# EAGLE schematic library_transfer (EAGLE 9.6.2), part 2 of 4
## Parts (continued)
Unconnected: A1.1(AUD_ON) A1.3(AF_OUT) A1.5(PTT) A1.6(PD) A1.7(H/L) A1.8(VIN) A1.9(GND) A1.10(GND) A1.12(ANT) A1.16(RXD) A1.17(TXD) A1.18(MIC_IN) A2.P$1(GND1) A2.P$2(MISO) A2.P$3(MOSI) A2.P$4(SCK) A2.P$5(NSS) A2.P$6(RST) A2.P$7(DIO5) A2.P$8(GND2) A2.P$9(ANT) A2.P$10(GND3) A2.P$11(DIO3) A2.P$12(DIO4) A2.P$13(3.3V) A2.P$14(DIO0) A2.P$15(DIO1) A2.P$16(DIO2) A3.1(VIN+) A3.2(VIN-) A3.4(VOUT-) A3.6(VOUT+) A4.1(1-2) A4.2(1-2) A4.3(3-4) A4.4(3-4) A4.6 A4.7 A4.8 ANT1.P$1(GND) ANT1.P$2(ANT) ANT1.P$3(GND) ANT2.IN1 ANT3.IN1 ANT3.IN2 B1.1(P) B1.2(M) B1.3(N) B2.1(N) B2.2(M) B2.3(P) B3.+ B3.- B4.+1 B4.+2 B4.-1 B4.-2 B5.+1(+) B5.+2(+) B5.- B6.+ B6.- B7.N(-) B7.P(+) B8.+1(+) B8.+2(+) B8.-1(-) B8.-2(-) B11.+ B11.- B12.+ B12.- B13.N B13.P B14.+ B14.- B15.+ B15.- B16.1 B16.2 B17.+1(+) B17.+2(+) B17.-1(-) B17.-2(-) C1.P$1 C1.P$2 C2.+ C2.- C3.+ C3.- C4.P$1 C4.P$2 C5.+ C5.- C6.+ C6.- C7.P$1 C7.P$2 C8.P$1 C8.P$2 C9.1 C9.2 C10.P$1 C10.P$2 C11.COLD C11.HOT C12.COLD C12.HOT C13.+1 C13.+2 C13.-1 C13.-2 C14.N(-) C14.P(+) C15.+ C15.- C16.N(-) C16.P(+) C17.N(-) C17.P(+) C18.1A C18.1B C18.2A C18.2B C19.P$1 C19.P$2 C20.+ C20.- C21.+ C21.- C22.1 C22.2 C23.1 C23.2 C24.1 C24.2 C25.P$1 C25.P$2 C26.1 C26.2 C27.1 C27.2 C28.P$1 C28.P$2 C29.+ C29.- C30.+ C30.- C31.N(-) C31.P(+) C32.P$1 C32.P$2 CM1.1(GND) CM1.2(EMMC_DISABLE_N) CM1.3(GPIO-00) CM1.4(SDX_VDD) CM1.5(GPIO-01) CM1.6(SDX_VDD) CM1.7(GND) CM1.8(GND) CM1.9(GPIO-02) CM1.10(SDX_CLK) CM1.11(GPIO-03) CM1.12(SDX_CMD) CM1.13(GND) CM1.14(GND) CM1.15(GPIO-04) CM1.16(SDX_D0) CM1.17(GPIO-05) CM1.18(SDX_D1) CM1.19(GND) CM1.20(GND) CM1.21(GPIO-06) CM1.22(SDX_D2) CM1.23(GPIO-07) CM1.24(SDX_D3) CM1.25(GND) CM1.26(GND) CM1.27(GPIO-08) CM1.28(GPIO-28) CM1.29(GPIO-09) CM1.30(GPIO-29) CM1.31(GND) CM1.32(GND) CM1.33(GPIO-10) CM1.34(GPIO-30) CM1.35(GPIO-11) CM1.36(GPIO-31) CM1.37(GND) CM1.38(GND) CM1.39(GPIO0-27_VDD) CM1.40(GPIO0-27_VDD) CM1.41(GPIO28-45_VDD) CM1.42(GPIO28-45_VDD) CM1.43(GND) CM1.44(GND) CM1.45(GPIO-12) CM1.46(GPIO-32) CM1.47(GPIO-13) CM1.48(GPIO-33) CM1.49(GND) CM1.50(GND) CM1.51(GPIO-14) CM1.52(GPIO-34) CM1.53(GPIO-15) CM1.54(GPIO-35) CM1.55(GND) CM1.56(GND) CM1.57(GPIO-16) CM1.58(GPIO-36) CM1.59(GPIO-17) CM1.60(GPIO-37) CM1.61(GND) CM1.62(GND) CM1.63(GPIO-18) CM1.64(GPIO-38) CM1.65(GPIO-19) CM1.66(GPIO-39) CM1.67(GND) CM1.68(GND) CM1.69(GPIO-20) CM1.70(GPIO-40) CM1.71(GPIO-21) CM1.72(GPIO-41) CM1.73(GND) CM1.74(GND) CM1.75(GPIO-22) CM1.76(GPIO-42) CM1.77(GPIO-23) CM1.78(GPIO-43) CM1.79(GND) CM1.80(GND) CM1.81(GPIO-24) CM1.82(GPIO-44) CM1.83(GPIO-25) CM1.84(GPIO-45) CM1.85(GND) CM1.86(GND) CM1.87(GPIO-26) CM1.88(HDMI_HPD_N_1V8) CM1.89(GPIO-27) CM1.90(EMMC_EB_N_1V8) CM1.91(GND) CM1.92(GND) CM1.93(DSI0_DN1) CM1.94(DSI1_DP0) CM1.95(DSI0_DP1) CM1.96(DSI1_DN0) CM1.97(GND) CM1.98(GND) CM1.99(DSI0_DN0) CM1.100(DSI1_CP) CM1.101(DSI0_DP0) CM1.102(DSI1_CN) CM1.103(GND) CM1.104(GND) CM1.105(DSI0_CN) CM1.106(DSI1_DP3) CM1.107(DSI0_CP) CM1.108(DSI1_DN3) CM1.109(GND) CM1.110(GND) CM1.111(HDMI_CLK_N) CM1.112(DSI1_DP2) CM1.113(HDMI_CLK_P) CM1.114(DSI1_DN2) CM1.115(GND) CM1.116(GND) CM1.117(HDMI_D0_N) CM1.118(DSI1_DP1) CM1.119(HDMI_D0_P) CM1.120(DSI1_DN1) CM1.121(GND) CM1.122(GND) CM1.123(HDMI_D1_N) CM1.124(NC) CM1.125(HDMI_D1_P) CM1.126(NC) CM1.127(GND) CM1.128(NC) CM1.129(HDMI_D2_N) CM1.130(NC) CM1.131(HDMI_D2_P) CM1.132(NC) CM1.133(GND) CM1.134(GND) CM1.135(CAM1_DP3) CM1.136(CAM0_DP0) CM1.137(CAM1_DN3) CM1.138(CAM0_DN0) CM1.139(GND) CM1.140(GND) CM1.141(CAM1_DP2) CM1.142(CAM0_CP) CM1.143(CAM1_DN2) CM1.144(CAM0_CN) CM1.145(GND) CM1.146(GND) CM1.147(CAM1_CP) CM1.148(CAM0_DP1) CM1.149(CAM1_CM) CM1.150(CAM0_DN1) CM1.151(GND) CM1.152(GND) CM1.153(CAM1_DP1) CM1.154(NC) CM1.155(CAM1_DN1) CM1.156(NC) CM1.157(GND) CM1.158(NC) CM1.159(CAM1_DP0) CM1.160(NC) CM1.161(CAM1_DN0) CM1.162(NC) CM1.163(GND) CM1.164(GND) CM1.165(USB_DP) CM1.166(TVDAC) CM1.167(USB_DN) CM1.168(USB_OTGID) CM1.169(GND) CM1.170(GND) CM1.171(HDMI_CEC) CM1.172(VC_TRST_N) CM1.173(HDMI_SDA) CM1.174(VC_TDI) CM1.175(HDMI_SCL) CM1.176(VC_TMS) CM1.177(RUN) CM1.178(VC_TDO) CM1.179(VDD_CORE_(DNC)) CM1.180(VC_TCK) CM1.181(GND) CM1.182(GND) CM1.183(1.8V) CM1.184(1.8V) CM1.185(1.8V) CM1.186(1.8V) CM1.187(GND) CM1.188(GND) CM1.189(VDAC) CM1.190(VDAC) CM1.191(3.3V) CM1.192(3.3V) CM1.193(3.3V) CM1.194(3.3V) CM1.195(GND) CM1.196(GND) CM1.197(VBATT) CM1.198(VBATT) CM1.199(VBATT) CM1.200(VBATT) CR1.A CR1.C(K) CR2.1(K) CR2.2(A) CR3.A CR3.C(K) CR4.1(A) CR4.2(A) CR4.3(K) CR5.1(A1) CR5.2(K) CR5.3(A2) CR6.1 CR6.3 CR6.TAB CR7.A CR7.K CR8.A CR8.K CR9.A CR9.C(K) CR10.A CR10.C(K) CR11.1(A1) CR11.3(A2) CR11.T(K) CR12.A CR12.K CR13.P$1 CR13.P$2 CR13.P$3 CR14.1 CR14.3 CR14.TAB CR15.1 CR15.2 CR15.3 CR16.A CR16.K CR17.A CR17.K CR18.1(K) CR18.2(A) CR19.1(K) CR19.2(A) CR20.A CR20.C(K) CR21.A CR21.C(K) CR22.A CR22.K D1.A1 D1.A2 D1.K1 D1.K2 D2.A D2.K D3.A D3.K1(K) D3.K2(K) D4.1(K) D4.3(A) D5.A D5.K D6.1(A) D6.2(K) D7.2(GND) D7.3(VCC) D7.4(IO2) D7.5(IO1) D8.1(A) D8.2(K) D8.3(COM) D9.A D9.C(K) D10.A D10.K D11.A D11.K D12.1(CC1) D12.2(E) D12.3(D) D12.4(C) D12.5(CC2) D12.6(B) D12.7(A) D12.8(DP) D12.9(F) D12.10(G) D13.A D13.K D14.1(K) D14.3(A) D15.1(A) D15.3(A) D15.T(K) D16.A D16.K D17.A D17.K D18.1(K) D18.2(A) D19.1(K) D19.2(A) D20.1(K) D20.2(A) D21.A D21.K1(K) D21.K2(K) D22.1(A) D22.2(A) D22.3(K) D23.A D23.K D24.A D24.K D25.1(REF) D25.2(K) D25.3(A) D26.1(A) D26.3(K) D27.A D27.K(C) D28.A D28.K D29.A D29.K(C) D30.A D30.K D31.A D31.K(C) D32.A D32.K D33.A D33.K D34.A D34.C(K) D35.A D35.K D36.1(K) D36.2(A) F1.P$1 F1.P$2 F2.P$1 F2.P$2 F3.P$1 F3.P$2 F4.P$1 F4.P$2 F5.P$1 F5.P$2 F6.P$1 F6.P$2 F7.P$1 F7.P$2 F8.1 F8.2(GND) F8.3(GND) F8.4 F8.5(GND) F9.P$1 F9.P$2 F10.1A F10.2A F10.3B F10.4B F13.P$1 F13.P$2 F14.P$1 F14.P$2 F15.P$1 F15.P$2 F16.P$1 F16.P$2 FB1.P$1 FB1.P$2 GDT1.P$1 GDT1.P$2 GDT2.P$1 GDT2.P$2 GDT3.C GDT3.L1 GDT3.L2 HS1.P$1 HS1.P$2 HS1.P$3 HS1.P$4 HS2.P$1 HS2.P$2 HS3.P$1 HS3.P$2 HS4.P$1 HS4.P$2 HS4.P$3 HS4.P$4 HS5.P$1 HS5.P$2 J1.1 J1.2 J1.3 J1.4 J2.N J2.P J3.+(P) J3.-(N) J4.+(P) J4.-(N) J5.N J5.P J6.+(P) J6.-(N) J7.A1(GND) J7.A4(VCC) J7.A5(CC1) J7.A6(D+) J7.A7(D-) J7.A8(SBV1) J7.A9(VCC) J7.A12(GND) J7.B1(GND) J7.B4(VCC) J7.B5(CC2) J7.B6(D+) J7.B7(D-) J7.B8(SBV2) J7.B9(VCC) J7.B12(GND) J8.A1(GND) J8.A4(VCC) J8.A5(CC1) J8.A6(D+) J8.A7(D-) J8.A8(SBV1) J8.A9(VCC) J8.A12(GND) J8.B1(GND) J8.B4(VCC) J8.B5(CC2) J8.B6(D+) J8.B7(D-) J8.B8(SBV2) J8.B9(VCC) J8.B12(GND) J9.A1(GND) J9.A4(VCC) J9.A5(CC1) J9.A6(D+) J9.A7(D-) J9.A8(SBV1) J9.A9(VCC) J9.A12(GND) J9.B1(GND) J9.B4(VCC) J9.B5(CC2) J9.B6(D+) J9.B7(D-) J9.B8(SBV2) J9.B9(VCC) J9.B12(GND) J10.1(VCC1) J10.2(D-1) J10.3(D+1) J10.4(GND1) J10.5(VCC2) J10.6(D-2) J10.7(D+2) J10.8(GND2) J10.G1(CASE1) J10.G2(CASE1) J10.G3(CASE2) J10.G4(CASE2) J11.1(VCC) J11.2(D-) J11.3(D+) J11.4(GND) J11.S1(CASE) J11.S2(CASE) J12.1(VCC) J12.2(D-) J12.3(D+) J12.4(GND) J12.MH1(CASE) J12.MH2(CASE) J13.1(NC1) J13.2(NC2) J13.3(IN) J13.4(NC4) J13.5(NC5) J13.6(CAP) J13.7(NC7) J13.8(NC8) J13.9(NC9) J13.10(OUT10) J13.11(OUT11) J13.12(NC12) J13.13(NC13) J13.14(NC14) J13.15(NC15) J13.16(NC16) J13.EP J14.1A J14.1B J14.2A J14.2B J14.3A J14.3B J15.1A J15.1B J15.2A J15.2B J16.G1(GND) J16.G2(GND) J16.G3(GND) J16.G4(GND) J16.S(RF) J17.G1(GND) J17.G2(GND) J17.G3(GND) J17.G4(GND) J17.RF J18.1(S) J18.2(T) J18.3(R) J19.R J19.S J19.T J20.1(S) J20.2(T) J20.3(R) J21.R J21.S J21.T J22.1(S) J22.2(T) J22.3(R1) J22.4(R2) J23.P$1 J23.P$2 J24.1 J24.2 J24.3 J24.4 J24.5 J24.6 J24.7 J24.8 J24.9 J24.10 J25.DND4(GND) J25.GND1(GND) J25.GND2(GND) J25.GND3(GND) J25.SIG(RF) J26.C1(VSS) J26.C2(VSS) J26.C3(VSS) J26.C4(VSS) J26.DSW1(SW1) J26.DSW2(SW2) J26.P1(DAT2) J26.P2(DAT3/CS) J26.P3(CMD/MOSI) J26.P4(VDD) J26.P5(CLK) J26.P6(VSS) J26.P7(DAT0/MISO) J26.P8(DAT1) J27.1(D2) J27.2(D3) J27.3(CMD) J27.4(VDD) J27.5(CLK) J27.6(VSS) J27.7(D0) J27.8(D1) J27.P$1(CASE) J27.P$2(CASE) J27.P$3(CASE) J27.P$4(CASE) J28.1 J28.2 J28.3 J28.4 J28.5 J28.6 J28.7 J28.8 J28.9 J28.10 J28.11 J28.12 J28.13 J28.14 J28.15 J29.1 J29.2 J29.3 J29.4 J29.5 J29.6 J29.7 J29.8 J29.9 J30.1A J30.1B J30.2A J30.2B J30.3A J30.3B J31.1A J31.1B J31.2A J31.2B J32.1(V+) J32.2(GND) J32.3(NO) J33.G1(GND) J33.G2(GND) J33.SIG(RF) J34.GND1(GND) J34.GND2(GND) J34.GND3(GND) J34.GND4(GND) J34.RF J35.1 J35.2 J35.3 J35.4 J35.5 J35.6 J35.7 J35.8 J35.9 J35.10 J35.11 J35.12 J35.13 J35.14 J35.15 J35.16 J36.1 J36.2 J36.3 J36.4 J36.MECH1(MT1) J36.MECH2(MT2) J37.P$1 J38.1 J38.2 J38.3 J38.4 J38.5 J39.1 J39.2 J39.3 J39.4 J39.5 J39.6 J39.7 J39.8 J39.9 J39.10 J39.11 J39.12 J39.13 J39.14 J39.15 J39.16 J39.17 J39.18 J39.19 J39.20 J39.21 J39.22 J39.23 J39.24 J39.25 J39.26 J39.27 J39.28 J39.29 J39.30 J39.31 J39.32 J39.33 J39.34 J39.35 J39.36 J39.37 J39.38 J39.39 J39.40 J40.1(VCC1) J40.2(D-1) J40.3(D+1) J40.4(GND1) J40.5(VCC2) J40.6(D-2) J40.7(D+2) J40.8(GND2) J40.P$9(CASE1) J40.P$10(CASE2) J40.P$11(CASE2) J40.P$12(CASE1) J41.1(VCC) J41.2(D-) J41.3(D+) J41.4(GND) J41.P$5(CASE) J41.P$6(CASE) J42.1(RTH_TCT) J42.2(ETH_TDP) J42.3(ETH_TDN) J42.4(ETH_RDP) J42.5(USB_RDN) J42.6(ETH_RCT) J42.13(RIGHT_LED_C) J42.14(RIGHT_LED_A) J42.15(LEFT_LED_C) J42.16(LEFT_LED_A) J42.P$5(SHIELD) J42.P$6(SHIELD) J42.P$7(SHIELD) J42.P$8(SHIELD) J42.P$9(SHIELD) J42.P$10(SHIELD) J42.U1(USB_VCC) J42.U2(USB_DM) J42.U3(USB_DP) J42.U4(USB_GND) J43.1(NC) J43.2(AGND) J43.3(SDA) J43.4(AVDD) J43.5(SCL) J43.6(RESET) J43.7(VS) J43.8(PWDN) J43.9(HS) J43.10(DVDD) J43.11(DOVDD) J43.12(D9) J43.13(MCLK) J43.14(D8) J43.15(DGND) J43.16(D7) J43.17(PCLK) J43.18(D6) J43.19(D2) J43.20(D5) J43.21(D3) J43.22(D4) J43.23(D1) J43.24(D0) J43.P$1(DGND) J43.P$2(DGND) J44.P$1 J45.1 J45.2 J45.3 J45.4 J45.5 J45.6 J45.7 J45.8 J45.9 J46.1 J46.2 J46.3 J46.4 J46.5 J46.6 J46.7 J46.8 J46.9 J47.1 J47.2 J47.3 J47.4 J47.5 J47.6 J47.7 J47.8 J47.S1 J47.S2 J49.1A J49.1B J49.2A J49.2B J50.1 J50.2 J51.1 J51.2 J51.3 J51.4 J51.5 J52.G1(GND) J52.G2(GND) J52.G3(GND) J52.G4(GND) J52.S(RF) J53.P$1(RF) J53.P$2(GND) J53.P$3(GND) J53.P$4(GND) J53.P$5(GND) J54.N(GND) J54.P(RF) J54.S1(GND) J54.S2(GND) J55.1 J55.2 J56.1 J56.2 J56.3 J56.4 J56.5 J56.6 J56.7 J56.8 J56.9 J56.10 J56.11 J56.12 J56.13 J56.14 J56.15 J56.16 J56.17 J56.18 J56.19 J56.20 J56.21 J56.22 J56.23 J56.24 J56.25 J56.26 J56.27 J56.28 J56.29 J56.30 J56.31 J56.32 J56.33 J56.34 J56.35 J56.36 J56.37 J56.38 J56.39 J56.40 J56.FN1(FN) J56.FN2(FN) J56.FN3(FN) J56.FN4(FN) J57.1 J57.2 J58.1A J58.1B J58.2A J58.2B J58.3A J58.3B J58.4A J58.4B J58.5A J58.5B J58.6A J58.6B J58.7A J58.7B J58.8A J58.8B J59.L J59.R J60.1 J60.2 J60.3 J61.1 J61.2 J61.3 J62.1(1VCC) J62.2(2DM) J62.3(3DP) J62.4(4ID) J62.5(5GND) J62.GND(CASE) J63.1 J63.2 J63.3 J63.4 J63.5 J63.6 J63.7 J63.8 J63.9 J63.10 J63.11 J63.12 J63.13 J63.14 J63.15 J63.16 J63.17 J63.18 J63.19 J63.20 J63.21 J63.22 J63.23 J63.24 J63.25 J63.26 J63.27 J63.28 J63.29 J63.30 J63.31 J63.32 J63.33 J63.34 J63.35 J63.36 J63.37 J63.38 J63.39 J63.40 J63.41 J63.42 J63.43 J63.44 J63.45 J63.46 J63.47 J63.48 J63.49 J63.50 J63.51 J63.52 J63.53 J63.54 J63.55 J63.56 J63.57 J63.58 J63.59 J63.60 J63.61 J63.62 J63.63 J63.64 J64.1 J64.2 J64.3 J64.4 J64.5 J64.M1(C) J64.M2(C) J64.M3(C) J64.M4(C) J65.1 J65.2 J65.3 J65.4 J65.5 J65.6 J65.7 J65.8 J65.S1 J65.S2 J66.G1(GND) J66.G2(GND) J66.G3(GND) J66.G4(GND) J66.RF J67.1 J67.2 J68.1 J68.2 J68.P1 J68.P2 J69.P$1 J70.RING J70.TIP J71.1 J71.2 J71.3 J71.4 J71.5 J71.6 J72.P$1 J72.P$2 J72.P$3 J72.P$4 J72.P$5 J72.P$6 J72.P$7 J72.P$8 J73.P$1 J73.P$2 J73.P$3 J73.P$4 J73.P$5 J73.P$6 J74.P$1 J74.P$2 J74.P$3 J74.P$4 J75.P$1 J75.P$2 J76.P$1 J77.P$1 J78.P$1 J78.P$2 J78.P$3 J78.P$4 J79.P$1 J79.P$2 J79.P$3 J79.P$4 J80.GND J80.L J80.N J81.1 J81.2 J81.3 J81.4 J81.5 J81.6 J81.7 J81.8 J81.9 J81.10 J81.11 J81.12 J81.13 J81.14 J82.1(SHIELD_2) J82.2(DATA_2_P) J82.3(DATA_2_N) J82.4(SHIELD_1) J82.5(DATA_1_P) J82.6(DATA_1_N) J82.7(SHIELD_0) J82.8(DATA_0_P) J82.9(DATA_0_N) J82.10(SHIELD_CLK) J82.11(CLK_P) J82.12(CLK_N) J82.13(GND) J82.14(CEC) J82.15(SCL) J82.16(SDA) J82.17(UTILITY) J82.18(+5V) J82.19(HPD) J82.P$1(GND) J82.P$2(GND) J82.P$3(GND) J82.P$4(GND) J83.1(BTM) J83.2(BTM) J83.3(TOP) J84.1 J84.2 J85.1 J85.2 J85.3 J85.4 J85.5 J85.6 J85.7 J85.8 J85.9 J85.10 J85.11 J85.12 J85.13 J85.14 J85.15 J85.16 J85.17 J85.18 J85.19 J85.20 J86.P$1 J86.P$2 J87.1 J87.2 J87.3 J87.4 J87.5 J87.6 J87.7 J87.8 J87.9 J87.10 J88.1 J88.2 J88.3 J88.4 J88.5 J88.6 J88.7 J88.8 J88.9 J88.10 L1.P$1 L1.P$2 L2.P$1 L2.P$2 L3.P$1 L3.P$2 L4.P$1 L4.P$2 L5.P$1 L5.P$2 L6.P$1 L6.P$2 L7.P$1 L7.P$2 L8.P$1 L8.P$2 L9.P$1 L9.P$2 L10.P$1 L10.P$2 L11.P$1 L11.P$2 L12.P$1 L12.P$2 L13.P$1 L13.P$2 L14.P$1 L14.P$2 L15.P$1 L15.P$2 L16.P$1 L16.P$2 L17.IN1(1IN) L17.IN2(2IN) L17.OUT1(1OUT) L17.OUT2(2OUT) L18.P$1 L18.P$2 L19.1 L19.2 L20.1 L20.2 L21.A1(1IN) L21.A2(1OUT) L21.B1(2IN) L21.B2(2OUT) L22.1 L22.2 L23.P$1 L23.P$2 L24.1(P+) L24.3(P-) L24.4(S+) L24.5(SCT) L24.6(S-) L25.P$1 L25.P$2 L26.P$1 L26.P$2 L27.P$1 L27.P$2 L28.P$1 L28.P$2 L29.P$1 L29.P$2 L30.P$1 L30.P$2 L31.P$1 L31.P$2 L32.P$1 L32.P$2 L33.P$1 L33.P$2 L34.P$1 L34.P$2 L35.P$1 L35.P$2 L36.P$1 L36.P$2 L37.P$1 L37.P$2 L38.P$1 L38.P$2 L39.P$1 L39.P$2 L40.P$1 L40.P$2 L41.IN1(1IN) L41.IN2(2IN) L41.OUT1(1OUT) L41.OUT2(2OUT) L42.1 L42.2 L43.1(1IN) L43.2(2IN) L43.3(1OUT) L43.4(2OUT) L44.P$1 L44.P$2 L45.P$1 L45.P$2 L46.1(1IN) L46.2(2IN) L46.3(2OUT) L46.4(1OUT) L47.P$1 L47.P$2 L48.1 L48.2 L49.1(1IN) L49.2(1OUT) L49.3(2OUT) L49.4(2IN) L50.1(1IN) L50.2(1OUT) L50.3(2OUT) L50.4(2IN) L51.P$1 L51.P$2 L52.P$1 L52.P$2 L53.P$1 L53.P$2 L54.P$1 L54.P$2 L55.P$1 L55.P$2 L56.P$1 L56.P$2 L57.P$1 L57.P$2 L58.1 L58.2 L59.1 L59.2 L60.P$1 L60.P$2 L61.P$1 L61.P$2 L62.1 L62.2 LS1.P$1 LS1.P$2 MOV1.P$1 MOV1.P$2 Q1.1(B) Q1.3(E) Q1.T(C) Q2.1(G) Q2.2(S) Q2.3(D) Q3.1(G) Q3.2(D) Q3.3(S) Q4.1(S) Q4.2(S) Q4.3(S) Q4.4(G) Q4.5(D) Q4.6(D) Q4.7(D) Q4.8(D) Q5.1(G) Q5.2(D) Q5.3(S) Q5.T(D) Q6.1(S) Q6.2(S) Q6.3(S) Q6.4(G) Q6.15(D) Q7.1_S(S) Q7.2_S(S) Q7.3_S(S) Q7.4_G(G) Q7.5_D(D) Q7.6_D(D) Q7.7_D(D) Q7.8_D(D) Q7.D Q8.1(S) Q8.2(S) Q8.3(S) Q8.4(G) Q8.15(D) Q10.1(G) Q10.3(S) Q10.TAB(D) Q11.D Q11.G Q11.S Q12.1(B) Q12.2(E) Q12.3(C) Q13.1(B) Q13.2(E) Q13.3(C) Q14.1(G) Q14.3(S) Q14.TAB(D) Q15.1(B) Q15.2(E) Q15.3(C) Q16.1(B) Q16.2(E) Q16.3(C) Q17.1(B) Q17.2(E) Q17.3(C) Q18.1(G) Q18.3(S) Q18.T(D) Q19.1(G) Q19.3(S) Q19.T(D) Q20.1(G) Q20.2(D) Q20.3(S) Q21.1(G) Q21.2(D) Q21.3(S) Q22.1(G) Q22.3(S) Q22.TAB(D) Q23.1(G) Q23.2(D) Q23.3(S) Q24.1(G) Q24.3(S) Q24.T(D) Q25.D Q25.G Q25.S Q26.1(S) Q26.2(S) Q26.3(S) Q26.4(G) Q26.5(D) Q26.6(D) Q26.7(D) Q26.8(D) Q26.P$1(D) Q27.1(S) Q27.2(S) Q27.3(S) Q27.4(G) Q27.5(D) Q27.6(D) Q27.7(D) Q27.8(D) Q27.8_P(D) Q28.1(S) Q28.2(G) Q28.3(D) Q28.4(S) Q28.5(G) Q28.6(D) Q29.1(G) Q29.2(D) Q29.3(S) Q29.4(S) Q29.5(D) Q29.6(D) Q29.7(S) Q29.8(S) Q29.9(D) Q29.10(D) Q29.11(S) Q29.12(S) Q29.13(D) Q29.14(D) Q29.15(S) Q29.16(S) Q29.17(D) Q29.18(D) Q29.19(S) Q29.20(S) Q29.21(D) Q29.22(D) Q29.23(S) Q29.24(S) Q29.25(D) Q29.26(D) Q29.27(S) Q29.28(S) Q29.29(D) Q29.30(D) Q30.1(G) Q30.2(S) Q30.3(D) Q31.D Q31.G Q31.S Q32.1(VIN) Q32.3(TG) Q32.4(TGR) Q32.5(BG) Q32.6(SW) Q32.7(SW) Q32.8(SW) Q32.TP(PGND) Q33.1(S) Q33.2(S) Q33.3(S) Q33.4(G) Q33.5(D) Q33.6(D) Q33.7(D) Q33.8(D) Q33.TP(D) Q34.1(D) Q34.2(D) Q34.3(G) Q34.4(S) Q34.5(D) Q34.6(D) Q34.7(S) Q34.8(D) Q35.1(G) Q35.2(D) Q35.3(S) Q35.T(D) Q36.D1(D) Q36.D2(D) Q36.D3(D) Q36.G Q36.S Q37.1(G) Q37.2(S) Q37.3(D) Q38.1(D) Q38.2(G) Q38.3(S) Q38.4(G) Q38.5(D) Q38.6(S) Q39.1(S) Q39.2(S) Q39.3(S) Q39.4(G) Q39.5(D) Q39.6(D) Q39.7(D) Q39.8(D) Q40.1(G) Q40.2(S) Q40.3(D) Q41.1(G) Q41.2(D) Q41.G(S) Q42.D Q42.G Q42.P$2(S) Q42.P$3(S) Q42.S Q43.D Q43.G Q43.S R1.1 R1.2 R2.1 R2.2(ADJ) R2.3 R3.1 R3.2(ADJ) R3.3 R4.1 R4.2 R4.3 R5.1 R5.2 R5.3 R6.1 R6.2 R6.3 R7.1 R7.2 R7.3 R8.1 R8.2 R8.3 R9.1 R9.2 R9.3 R9.S1 R9.S2 R10.P$1 R10.P$2 R11.1 R11.2 R11.3 R12.1 R12.2 R13.1 R13.2 R14.1 R14.2 R15.1 R15.2 RT1.1 RT1.2 S2.1 S2.7 S2.8(NO) S2.9(GND) S2.10(GND) S2.11(COM) S2.12(GND) S2.13(GND) S2.14(NC) S3.P$1 S3.P$2 S3.P$3 S3.P$4 S3.P$5 S3.P$6 S3.P$7 S3.P$8 S3.P$9 S3.P$10 S3.P$11 S3.P$12 S3.P$13 S3.P$14 S3.P$15 S3.P$16 S3.P$17 S3.P$18 S3.P$19 S3.P$20 S3.P$21 S3.P$22 S3.P$23 S3.P$24 S3.P$25 S3.P$26 S3.P$27 S3.P$28 SH1.P$1 SH1.P$2 SH1.P$3 SH1.P$4 SH1.P$5 SH1.P$6 SH1.P$7 SH1.P$8 SH1.P$9 SH1.P$10 SH1.P$11 SH1.P$12 SW1.1 SW1.2 SW1.3 SW1.4 SW1.C SW2.1 SW2.2 SW2.A SW2.B SW2.C SW3.S1 SW3.S2 SW4.SW1 SW4.SW2 SW5.1 SW5.2 SW5.3 SW5.4 SW5.5 SW5.7 SW5.8 SW5.9 SW5.10 SW5.11 SW5.A SW5.B SW6.C(COM) SW6.L SW6.R SW7.1 SW7.2(COM) SW7.3 SW8.C(COM) SW8.L SW8.R SW9.1 SW9.2 SW9.C(COM) SW10.1 SW10.2 SW10.3 SW10.4 SW10.5 SW10.6 T1.P$1 T3.1(OUT+) T3.2(GND2) T3.3(OUT-) T3.4(IN) T3.5(GND1) T4.1(1P_PHY) T4.2(1C_PHY) T4.3(1N_PHY) T4.6(2P_PHY) T4.7(2C_PHY) T4.8(2N_PHY) T4.9(2N) T4.10(2C) T4.11(2P) T4.14(1N) T4.15(1C) T4.16(1P) T5.1 T5.2 T5.3 T5.4 T5.5 T5.6 T6.1IN T6.1OUT T6.2IN T6.2OUT T7.1B T7.1F T7.2B T7.2F T8.1 T8.2 T8.3 T8.4 T8.5 T8.6 T9.1 T9.2 T9.3 T9.4 T9.5 T9.6 TP1.P$1 TP2.P$1 TP3.P$1 TP4.P$1 U1.1(V+) U1.2(IN) U1.3(GND) U1.4(SINK) U1.5(IN) U1.6(SOURCE) U2.1(GND) U2.2(OUT) U2.3(IN) U3.1(GND) U3.2(OUT) U3.3(IN) U4.1(GND1) U4.2(VCC) U4.3(DIO13/DOUT) U4.4(DIN/DIO14) U4.5(DIO12) U4.6(!RESET) U4.7(DIO10/RSSI) U4.8(DIO11/PWM1) U4.9(RSVD1) U4.10(DIO8/!DTR) U4.11(GND2) U4.12(DIO19/!SPI_ATTN) U4.13(GND3) U4.14(DIO18/SPI_CLK) U4.15(DIO17/!SPI_SS) U4.16(DIO16/SPI_MOSI) U4.17(DIO15/SPI_MISO) U4.18(RSVD2) U4.19(RSVD3) U4.20(RSVD4) U4.21(RSVD5) U4.22(GND4) U4.23(RSVD6) U4.24(DIO4) U4.25(DIO7/!CTS) U4.26(DIO9/!SLEEP) U4.27(VREF) U4.28(DIO5/ASSOC) U4.29(DIO6/!RTS) U4.30(DIO3/AD3) U4.31(DIO2/AD2) U4.32(DIO1/AD1) U4.33(DIO0/AD0) U4.34(RSVD7) U4.35(GND5) U4.36(RF) U4.37(RSVD8) U4.38(GND_PAD) U5.1(RST) U5.2(MISO) U5.3(MOSI) U5.4(SCK) U5.5(NSS) U5.6(VCC) U5.7(GND1) U5.8(NC) U5.9(GND2) U5.10(DIO1) U5.11(BUSY) U5.12(GND3) U5.13(GND4) U5.14(ANT) U6.1(+VIN) U6.2(ON/OFF) U6.3(-VIN) U6.4(-VOUT) U6.5(-SENSE) U6.6(TRIM) U6.7(+SENSE) U6.8(+VOUT) U7.1(IO1) U7.2(GND) U7.3(I02) U7.4(IO3) U7.5(VBUS) U7.6(IO4) U8.1(IN1) U8.2(IN2) U8.3(IN3) U8.4(IN4) U8.5(IN5) U8.6(IN6) U8.7(IN7) U8.8(GND) U8.9(VCC) U8.10(OUT7) U8.11(OUT6) U8.12(OUT5) U8.13(OUT4) U8.14(OUT3) U8.15(OUT2) U8.16(OUT1) U9.1(VDD) U9.2(GND) U9.3(IN+) U9.4(IN-) U9.5(OUT) U10.1(VDD) U10.2(HB) U10.3(HO) U10.4(HS) U10.5(HI) U10.6(LI) U10.7(VSS) U10.8(LO) U10.TP(VSS) U11.1(VCC) U11.2(OUT) U11.3(GND) U11.4(NC) U12.1(VCC) U12.2(X+) U12.3(Y+) U12.4(X-) U12.5(Y-) U12.6(GND) U12.7(VBAT) U12.8(AUX) U12.9(VREF) U12.10(IOVDD) U12.11(!PENIRQ) U12.12(DOUT) U12.13(BUSY) U12.14(DIN) U12.15(!CS) U12.16(DCLK) U13.1(OUT) U13.2(IN-) U13.3(IN+) U13.4(-VS) U13.5(IN+) U13.6(IN-) U13.7(OUT) U13.8(+VS) U14.1(NO) U14.2(GND) U14.3(NC) U14.4(COM) U14.5(VCC) U14.6(IN) U15.1(NO) U15.2(GND) U15.3(NC) U15.4(COM) U15.5(VCC) U15.6(IN) U16.1(IN) U16.2(GND) U16.3(EN) U16.5(OUT) U17.1(VOUT) U17.2(L2) U17.3(PGND) U17.4(L1) U17.5(VIN) U17.6(EN) U17.7(PS/SYNC) U17.8(VINA) U17.9(GND) U17.10(FB) U17.PG1(PGND) U17.PG2(PGND) U17.PG3(PGND) U17.PG4(PGND) U17.PG(PGND) U18.1(SW) U18.2(SW) U18.3(SW) U18.4(PG) U18.5(FB) U18.6(AGND) U18.7(FSW) U18.8(DEF) U18.9(SS) U18.10(AVIN) U18.11(PVIN) U18.12(PVIN) U18.13(EN) U18.14(VOS) U18.15(PGND) U18.16(PGND) U18.EP(PGND) U19.1(VIN) U19.2(CTRL) U19.3(SW) U19.4(GND) U19.5(COMP) U19.6(FB) U20.1(FSW) U20.2(VCC) U20.3(FB) U20.4(COMP) U20.5(GND) U20.6(VOUT) U20.7(EN) U20.8(ILIM) U20.9(VIN) U20.10(BOOT) U20.11(SW) U21.1(FB) U21.2(EN) U21.3(VIN) U21.4(GND) U21.5(SW) U21.6(VOUT) U22.1(VIN1) U22.2(VBST1) U22.3(SW1) U22.4(PGND1) U22.5(EN1) U22.6(SS1) U22.7(VFB1) U22.8(GND) U22.9(VREG5) U22.10(VFB2) U22.11(SS2) U22.12(EN2) U22.13(PGND2) U22.14(SW2) U22.15(VBST2) U22.16(VIN2) U22.P$1(GND) U23.1(VTX) U23.2(CC1) U23.3(CC2) U23.4(GND) U23.5(HIPWR) U23.6(CTL1) U23.7(CTL2) U23.8(CTL3) U23.11(!ENSRC) U23.12(PSEL) U23.13(DVDD) U23.14(PCTRL) U23.15(!GD) U23.16(VAUX) U23.17(VDD) U23.18(AGND) U23.19(ISNS) U23.20(VPWR) U23.21(VBUS) U23.22(GDNG) U23.23(GDNS) U23.24(DSCG) U23.EP(GND) U24.1(VTX) U24.2(CC1) U24.3(CC2) U24.4(GND) U24.5(HIPWR) U24.6(CTL1) U24.7(CTL2) U24.8(!EN12V/EN9V) U24.11(!UFP) U24.12(PSEL) U24.13(DVDD) U24.14(PCTRL) U24.15(!GD) U24.16(VAUX) U24.17(VDD) U24.18(AGND) U24.19(ISNS) U24.20(VPWR) U24.21(VBUS) U24.22(GDNG) U24.23(GDNS) U24.24(DSCG) U24.EP(GND) U25.1(IN) U25.2(GND) U25.3(EN) U25.4(!FAULT) U25.5(ILIM) U25.6(OUT) U26.1(DP1) U26.2(GND) U26.3(DP2) U26.4(DM2) U26.5(IN) U26.6(DM1) U27.1(OUT) U27.2(GND) U27.3(!FLT) U27.4(EN) U27.5(IN) U28.1(GND) U28.2(IN) U28.3(IN) U28.4(EN1) U28.5(EN2) U28.6(!FLT2) U28.8(OUT2) U28.9(OUT1) U28.10(!FLT1) U28.GF2(GND) U28.GF3(GND) U28.GF(GND) U29.1(OUT) U29.2(FB) U29.3(PG) U29.4(GND) U29.5(EN) U29.7(DELAY) U29.8(IN) U30.1(OUT) U30.2(-VS) U30.3(IN+) U30.4(IN-) U30.5(EN) U30.6(+VS) U31.1(OUT) U31.2(IN-) U31.3(IN+) U31.4(-VS) U31.5(IN+) U31.6(IN-) U31.7(OUT) U31.8(+VS) U32.1(AVDD) U32.2(AREG) U32.3(VREF) U32.4(AVSS) U32.5(MICBIAS) U32.6(INP1) U32.7(INM1) U32.8(INP2) U32.9(INM2) U32.10(INP3) U32.11(INM3) U32.12(INP4) U32.13(INM4) U32.14(SHDNZ) U32.15(ARRD1) U32.16(ADDR0) U32.17(SCL) U32.18(SDA) U32.19(IOVDD) U32.20(GPIO1) U32.21(SDOUT) U32.22(BLCK) U32.23(FSYNC) U32.24(DREG) U32.EP(VSS) U33.1(IVCC) U33.2(SWO) U33.3(SGND) U33.4(SWCS) U33.5(SS) U33.6(FB) U33.7(NC1) U33.8(COMP) U33.9(NC2) U33.10(SYNC) U33.11(FREQ) U33.12(GND) U33.13(EN) U33.14(IN) U33.T(GNDT) U34.2(TRIG) U34.3(OUT) U34.4(RESET) U34.5(CV) U34.6(TRSH) U34.7(DISCH) U35.2(CAP+) U35.3(GND) U35.4(CAP-) U35.5(VOUT) U35.6(LV) U35.7(OSC) U35.8(VIN) U36.1(VIN) U36.2(GND) U36.3(EN) U36.4(FB) U36.5(OUT) U37.1(GND) U37.2 U37.3(GND) U37.4(GND) U37.5(GND) U37.6 U37.7(GND) U37.8(GND) U38.1(RFI_LF) U38.5(XTA) U38.6(XTB) U38.7(NRESET) U38.8(DIO0) U38.9(DIO1/DCLK) U38.10(DIO2/DATA) U38.11(DIO3) U38.12(DIO4) U38.13(DIO5) U38.16(SCK) U38.17(MISO) U38.18(MOSI) U38.19(NSS) U38.20(RXTX/RF_MOD) U38.21(RFI_HF(GND)) U38.22(RFO_HF(GND)) U38.27(PA_BOOST) U38.28(RFO_LF) U39.1(GND) U39.2(MISO) U39.3(MOSI) U39.4(SCK) U39.5(NSS) U39.6(RST) U39.8(GND) U39.9(ANT) U39.10(GND) U39.11(RXE) U39.13(VCC) U39.15(DIO1) U39.16(BUSY) U40.1(VDD_IN) U40.2(GND1) U40.3(XTA) U40.4(XTB) U40.5(GND2) U40.6(DIO3) U40.7(VREG) U40.8(GND3) U40.9(DCDC_SW) U40.10(VBAT) U40.11(VBAT_IO) U40.12(DIO2) U40.13(DIO1) U40.14(BUSY) U40.15(NRST) U40.16(MISO) U40.17(MOSI) U40.18(SCK) U40.19(NSS) U40.20(GND4) U40.21(RFI_P) U40.22(RFI_N) U40.23(RFO) U40.24(VR_PA) U40.EP U41.1(CC1DB) U41.2(CC1) U41.3(NC) U41.4(CC2) U41.5(CC2DB) U41.6(RESET) U41.7(SCL) U41.8(SDA) U41.9(DISCH) U41.10(GND) U41.11(ATTACH) U41.12(ADDR0) U41.13(ADDR1) U41.14(POWER_OK3) U41.15(GPIO) U41.16(VBUS_EN_SNK) U41.17(A_B_SIDE) U41.18(VBUS_VS_DSICH) U41.19(ALERT#) U41.20(POWER_OK2) U41.21(VREG_1V2) U41.22(VSYS) U41.23(VREG_2V7) U41.24(VDD) U41.EP(EXPPAD) U42.1(PE2) U42.2(PE3) U42.3(PE4) U42.4(PE5) U42.5(PE6) U42.6(VBAT) U42.7(PI8) U42.8(PC13) U42.9(PC14) U42.10(PC15) U42.11(PI9) U42.12(PI10) U42.13(PI11) U42.14(VSS1) U42.15(VDD1) U42.16(PF0) U42.17(PF1) U42.18(PF2) U42.19(PI12) U42.20(PI13) U42.21(PI14) U42.22(PF3) U42.23(PF4) U42.24(PF5) U42.25(VSS2) U42.26(VDD2) U42.27(PF6) U42.28(PF7) U42.29(PF8) U42.30(PF9) U42.31(PF10) U42.32(PH0) U42.33(PH1) U42.34(NRST) U42.35(PC0) U42.36(PC1) U42.37(PC2) U42.38(PC3) U42.39(VDD3) U42.40(VSSA) U42.41(VREF+) U42.42(VDDA) U42.43(PA0) U42.44(PA1) U42.45(PA2) U42.46(PH2) U42.47(PH3) U42.48(PH4) U42.49(PH5) U42.50(PA3) U42.51(VSS3) U42.52(VDD4) U42.53(PA4) U42.54(PA5) U42.55(PA6) U42.56(PA7) U42.57(PC4) U42.58(PC5) U42.59(VDD5) U42.60(VSS4) U42.61(PB0) U42.62(PB1) U42.63(PB2) U42.64(PI15) U42.65(PJ0) U42.66(PJ1) U42.67(PJ2) U42.68(PJ3) U42.69(PJ4) U42.70(PF11) U42.71(PF12) U42.72(VSS5) U42.73(VDD6) U42.74(PF13) U42.75(PF14) U42.76(PF15) U42.77(PG0) U42.78(PG1) U42.79(PE7) U42.80(PE8) U42.81(PE9) U42.82(VSS6) U42.83(VDD7) U42.84(PE10) U42.85(PE11) U42.86(PE12) U42.87(PE13) U42.88(PE14) U42.89(PE15) U42.90(PB10) U42.91(PB11) U42.92(VCAP_1) U42.93(VSS7) U42.94(VDD8) U42.95(PJ5) U42.96(PH6) U42.97(PH7) U42.98(PH8) U42.99(PH9) U42.100(PH10) U42.101(PH11) U42.102(PH12) U42.103(VDD9) U42.104(PB12) U42.105(PB13) U42.106(PB14) U42.107(PB15) U42.108(PD8) U42.109(PD9) U42.110(PD10) U42.111(PD11) U42.112(PD12) U42.113(PD13) U42.114(VSS8) U42.115(VDD10) U42.116(PD14) U42.117(PD15) U42.118(VDDDSI) U42.119(VCAPDSI) U42.120(DSI_D0P) U42.121(DSI_D0N) U42.122(VSSDSI1) U42.123(DSI_CKP) U42.124(DSI_CKN) U42.125(VDD12DSI) U42.126(DSI_D1P) U42.127(DSI_D1N) U42.128(VSSDSI2) U42.129(PG2) U42.130(PG3) U42.131(PG4) U42.132(PG5) U42.133(PG6) U42.134(PG7) U42.135(PG8) U42.136(VSS9) U42.137(VDDUSB) U42.138(PC6) U42.139(PC7) U42.140(PC8) U42.141(PC9) U42.142(PA8) U42.143(PA9) U42.144(PA10) U42.145(PA11) U42.146(PA12) U42.147(PA13) U42.148(VCAP_2) U42.149(VSS10) U42.150(VDD11) U42.151(PH13) U42.152(PH14) U42.153(PH15) U42.154(PI0) U42.155(PI1) U42.156(PI2) U42.157(PI3) U42.158(VDD12) U42.159(PA14) U42.160(PA15) U42.161(PC10) U42.162(PC11) U42.163(PC12) U42.164(PD0) U42.165(PD1) U42.166(PD2) U42.167(PD3) U42.168(PD4) U42.169(PD5) U42.170(VSS11) U42.171(VDDSDMMC) U42.172(PD6) U42.173(PD7) U42.174(PJ12) U42.175(PJ13) U42.176(PJ14) U42.177(PJ15) U42.178(PG9) U42.179(PG10) U42.180(PG11) U42.181(PG12) U42.182(PG13) U42.183(PG14) U42.184(VSS12) U42.185(VDD13) U42.186(PK3) U42.187(PK4) U42.188(PK5) U42.189(PK6) U42.190(PK7) U42.191(PG15) U42.192(PB3) U42.193(PB4) U42.194(PB5) U42.195(PB6) U42.196(PB7) U42.197(BOOT0) U42.198(PB8) U42.199(PB9) U42.200(PE0) U42.201(PE1) U42.202(VSS13) U42.203(PDR_ON) U42.204(VDD14) U42.205(PI4) U42.206(PI5) U42.207(PI6) U42.208(PI7) U43.P$1(PE2) U43.P$2(PE3) U43.P$3(PE4) U43.P$4(PE5) U43.P$5(PE6) U43.P$6(VBAT) U43.P$7(PC13) U43.P$8(PC14) U43.P$9(PC15) U43.P$10(PF0) U43.P$11(PF1) U43.P$12(PF2) U43.P$13(PF3) U43.P$14(PF4) U43.P$15(PF5) U43.P$16(VSS1) U43.P$17(VDD1) U43.P$18(PF6) U43.P$19(PF7) U43.P$20(PF8) U43.P$21(PF9) U43.P$22(PF10) U43.P$23(PH0) U43.P$24(PH1) U43.P$25(NRST) U43.P$26(PC0) U43.P$27(PC1) U43.P$28(PC2) U43.P$29(PC3) U43.P$30(VDD2) U43.P$31(VSSA) U43.P$32(VREF+) U43.P$33(VDDA) U43.P$34(PA0) U43.P$35(PA1) U43.P$36(PA2) U43.P$37(PA3) U43.P$38(VSS2) U43.P$39(VDD3) U43.P$40(PA4) U43.P$41(PA5) U43.P$42(PA6) U43.P$43(PA7) U43.P$44(PC4) U43.P$45(PC5) U43.P$46(PB0) U43.P$47(PB1) U43.P$48(PB2) U43.P$49(PF11) U43.P$50(PF12) U43.P$51(VSS3) U43.P$52(VDD4) U43.P$53(PF13) U43.P$54(PF14) U43.P$55(PF15) U43.P$56(PG0) U43.P$57(PG1) U43.P$58(PE7) U43.P$59(PE8) U43.P$60(PE9) U43.P$61(VSS4) U43.P$62(VDD5) U43.P$63(PE10) U43.P$64(PE11) U43.P$65(PE12) U43.P$66(PE13) U43.P$67(PE14) U43.P$68(PE15) U43.P$69(PB10) U43.P$70(PB11) U43.P$71(VCAP_1) U43.P$72(VDD6) U43.P$73(PB12) U43.P$74(PB13) U43.P$75(PB14) U43.P$76(PB15) U43.P$77(PD8) U43.P$78(PD9) U43.P$79(PD10) U43.P$80(PD11) U43.P$81(PD12) U43.P$82(PD13) U43.P$83(VSS5) U43.P$84(VDD7) U43.P$85(PD14) U43.P$86(PD15) U43.P$87(PG2) U43.P$88(PG3) U43.P$89(PG4) U43.P$90(PG5) U43.P$91(PG6) U43.P$92(PG7) U43.P$93(PG8) U43.P$94(VSS6) U43.P$95(VDDUSB) U43.P$96(PC6) U43.P$97(PC7) U43.P$98(PC8) U43.P$99(PC9) U43.P$100(PA8) U43.P$101(PA9) U43.P$102(PA10) U43.P$103(PA11) U43.P$104(PA12) U43.P$105(PA13) U43.P$106(VCAP_2) U43.P$107(VSS7) U43.P$108(VDD8) U43.P$109(PA14) U43.P$110(PA15) U43.P$111(PC10) U43.P$112(PC11) U43.P$113(PC12) U43.P$114(PD0) U43.P$115(PD1) U43.P$116(PD2) U43.P$117(PD3) U43.P$118(PD4) U43.P$119(PD5) U43.P$120(VSS8) U43.P$121(VDDSDMMC) U43.P$122(PD6) U43.P$123(PD7) U43.P$124(PG9) U43.P$125(PG10) U43.P$126(PG11) U43.P$127(PG12) U43.P$128(PG13) U43.P$129(PG14) U43.P$130(VSS9) U43.P$131(VDD9) U43.P$132(PG15) U43.P$133(PB3) U43.P$134(PB4) U43.P$135(PB5) U43.P$136(PB6) U43.P$137(PB7) U43.P$138(BOOT0) U43.P$139(PB8) U43.P$140(PB9) U43.P$141(PE0) U43.P$142(PE1) U43.P$143(PDR_ON) U43.P$144(VDD10) U44.1(VBATT) U44.2(PC13) U44.3(PC14) U44.4(PC15) U44.5(OSCIN) U44.6(OSCOUT) U44.7(NRST) U44.8(GND_A) U44.9(VDD_A) U44.10(PA0) U44.11(PA1) U44.12(PA2) U44.13(PA3) U44.14(PA4) U44.15(PA5) U44.16(PA6) U44.17(PA7) U44.18(PB0) U44.19(PB1) U44.20(PB2/BOOT1) U44.21(PB10) U44.22(PB11) U44.23(GND) U44.24(VDD) U44.25(PB12) U44.26(PB13) U44.27(PB14) U44.28(PB15) U44.29(PA8) U44.30(PA9) U44.31(PA10) U44.32(PA11) U44.33(PA12) U44.34(SWIO) U44.35(GND) U44.36(VDD) U44.37(SWCLK) U44.38(PA15) U44.39(PB3) U44.40(PB4) U44.41(PB5) U44.42(PB6) U44.43(PB7) U44.44(BOOT0) U44.45(PB8) U44.46(PB9) U44.47(GND) U44.48(VDD) U45.1(1B) U45.2(1A) U45.3(1R) U45.4(~RE) U45.5(2R) U45.6(2A) U45.7(2B) U45.8(GND) U45.9(2D) U45.10(2Y) U45.11(2Z) U45.12(DE) U45.13(1Z) U45.14(1Y) U45.15(1D) U45.16(VCC) U46.1(Y0) U46.2(GND) U46.3(Y1) U46.4(COM) U46.5(VCC) U46.6(SEL) U47.1(RO) U47.2(!RE) U47.3(DE) U47.4(DI) U47.5(GND) U47.6(A) U47.7(B) U47.8(VCC) U48.1(VINA) U48.2(EN) U48.3(FB) U48.4(AGND) U48.5(NC) U48.6(VINSW) U48.7(SW) U48.8(PGND) U48.P$1(PGND) U49.1(-VIN) U49.2(+VIN) U49.3(RC) U49.6(+VOUT) U49.7(-VOUT) U50.1(VCC) U50.2(R) U50.3(D) U50.4(GND) U50.5(Y) U50.6(Z) U50.7(B) U50.8(A) U51.1(A) U51.2(B) U51.3(C) U51.4(!G2A) U51.5(!G2B) U51.6(G1) U51.7(Y7) U51.8(GND) U51.9(Y6) U51.10(Y5) U51.11(Y4) U51.12(Y3) U51.13(Y2) U51.14(Y1) U51.15(Y0) U51.16(VCC) U52.2(IN) U52.3(GND) U52.4(OUT) U52.6(VCC) U53.1(B:2Y0) U53.2(B:2Y2) U53.3(B:2COM) U53.4(B:2Y3) U53.5(B:2Y1) U53.6(A:INH) U53.7(B:GND) U53.8(B:GND) U53.9(A:B) U53.10(A:A) U53.11(A:1Y3) U53.12(A:1Y0) U53.13(A:1COM) U53.14(A:1Y1) U53.15(A:1Y2) U53.16(B:VCC) U54.1(Y4) U54.2(Y6) U54.3(COM) U54.4(Y7) U54.5(Y5) U54.6(INH) U54.7(GND) U54.8(GND) U54.9(C) U54.10(B) U54.11(A) U54.12(Y3) U54.13(Y0) U54.14(Y1) U54.15(Y2) U54.16(VCC) U55.1(I0) U55.2(I1) U55.3(O) U55.4(I0) U55.5(I1) U55.6(O) U55.7(V-) U55.8(O) U55.9(I0) U55.10(I1) U55.11(O) U55.12(I0) U55.13(I1) U55.14(V+) U56.1(A) U56.2(B) U56.3(QA) U56.4(QB) U56.5(QC) U56.6(QD) U56.7(GND) U56.8(CLK) U56.9(!CLR) U56.10(QE) U56.11(QF) U56.12(QG) U56.13(QH) U56.14(VCC) U57.1(D) U57.2(GND) U57.3(VCC) U57.4(R) U57.5(VREF) U57.6(CANL) U57.7(CANH) U57.8(RS) U58.1(B1) U58.2(A1) U58.3(R1) U58.4(1DE) U58.5(R2) U58.6(A2) U58.7(B2) U58.8(GND) U58.9(D2) U58.10(Y2) U58.11(Z2) U58.12(2DE) U58.13(Z1) U58.14(Y1) U58.15(D1) U58.16(VCC) U58.TP(GND) U59.1(B1) U59.2(A1) U59.3(R1) U59.4(1DE) U59.5(R2) U59.6(A2) U59.7(B2) U59.8(GND) U59.9(D2) U59.10(Y2) U59.11(Z2) U59.12(2DE) U59.13(Z1) U59.14(Y1) U59.15(D1) U59.16(VCC) U59.TP(GND) U60.1(GND) U60.2(RF1) U60.3(GND) U60.4(GND) U60.5(RF3) U60.6(GND) U60.7(CTRL) U60.8(EN) U60.9(VDD) U60.10(GND) U60.11(RF2) U60.12(GND) U60.P(GND) U61.1(GND) U61.2(RFC) U61.3(GND) U61.4(GND) U61.5(RF4) U61.6(GND) U61.7(RF3) U61.8(V1) U61.9(V2) U61.10(VDD) U61.11(GND) U61.12(RF2) U61.13(GND) U61.14(RF1) U61.P$13(GND) U62.1(RF1) U62.2(GND) U62.4(V1) U62.5(V2) U62.6(VDD) U62.7(GND) U62.8(GND) U62.9(RF2) U62.10(GND) U62.11(RFC) U62.12(GND) U62.P(GND) U63.1(GND) U63.2(RF1(C)) U63.3(GND) U63.4(GND) U63.5(RF3) U63.6(GND) U63.7(CTRL) U63.8(ENABLE) U63.9(VBATT) U63.10(GND) U63.11(RF2) U63.12(GND) U63.P(GND) U64.1(S) U64.2(T) U64.3(R) U65.1(VCIN) U65.2(PGOOD) U65.3(EN) U65.4(BOOT) U65.5(PHASE) U65.6(PHASE) U65.7(VIN) U65.8(VIN) U65.9(PGND) U65.10(PGND) U65.11(PGND) U65.12(SW) U65.13(SW) U65.14(SW) U65.16(VDRV) U65.17(PGND) U65.19(SS) U65.20(VOUT) U65.22(VFB) U65.23(AGND) U65.24(FSW) U65.25(ILIM) U65.26(VDD) U65.27(MODE) U65.AGND U65.PGND U65.PGND2(PGND) U65.SW U65.VIN U66.1(VDDA) U66.2(A1) U66.3(A2) U66.4(A3) U66.5(A4) U66.6(A5) U66.7(A6) U66.8(GNDA) U66.9(GNDB) U66.10(B6) U66.11(B5) U66.12(B4) U66.13(B3) U66.14(B2) U66.15(B1) U66.16(VDDB) U67.1(SDN) U67.2(RXP) U67.3(RXN) U67.4(TX) U67.6(VDD) U67.7(TXRAMP) U67.8(VDD) U67.9(GPIO0) U67.10(GPIO1) U67.11(NIRQ) U67.12(SCLK) U67.13(SDO) U67.14(SDI) U67.15(NSEL) U67.16(XOUT) U67.17(XIN) U67.18(GND) U67.19(GPIO2) U67.20(GPIO3) U67.CENTER(GND) U68.1(SDA) U68.2(SCL) U68.3(VCC) U68.4(GND) U69.1(BS) U69.2(GND) U69.3(FB) U69.4(EN) U69.5(VIN) U69.6(SW) U70.2(GPIO0) U70.3(GPIO1) U70.4(GPIO2) U70.5(GPIO3) U70.6(GPIO4) U70.7(GPIO5) U70.8(GPIO6) U70.9(GPIO7) U70.11(GPIO8) U70.12(GPIO9) U70.13(GPIO10) U70.14(GPIO11) U70.15(GPIO12) U70.16(GPIO13) U70.17(GPIO14) U70.18(GPIO15) U70.19(TESTEN) U70.20(XIN) U70.21(XOUT) U70.24(SWCLK) U70.25(SWD) U70.26(RUN) U70.27(GPIO16) U70.28(GPIO17) U70.29(GPIO18) U70.30(GPIO19) U70.31(GPIO20) U70.32(GPIO21) U70.34(GPIO22) U70.35(GPIO23) U70.36(GPIO24) U70.37(GPIO25) U70.38(GPIO26/ADC0) U70.39(GPIO27/ADC1) U70.40(GPIO28/ADC2) U70.41(GPIO29/ADC3) U70.44(VREG_VIN) U70.45(VREG_VOUT) U70.46(USB_DM) U70.47(USB_DP) U70.51(QSPI_SD3) U70.52(QSPI_SCLK) U70.53(QSPI_SD0) U70.54(QSPI_SD2) U70.55(QSPI_SD1) U70.56(QSPI_CSN) U71.1(ANT) U71.2(GND) U71.3(DIO3) U71.4(DIO4) U71.5(VCC) U71.6(DIO0) U71.7(DIO1) U71.8(DIO2) U71.9(3V3) U71.10(MISO) U71.11(MOSI) U71.12(SCK) U71.13(SS) U71.14(RST) U71.15(DIO5) U71.16(GND) U71.17(GND) U72.1(-VIN) U72.2(+VIN) U72.3(-VOUT) U72.4(+VOUT) U73.1(GP0) U73.2(GP1) U73.4(GP2) U73.5(GP3) U73.6(GP4) U73.7(GP5) U73.9(GP6) U73.10(GP7) U73.11(GP8) U73.12(GP9) U73.14(GP10) U73.15(GP11) U73.16(GP12) U73.17(GP13) U73.19(GP14) U73.20(GP15) U73.21(GP16) U73.22(GP17) U73.24(GP18) U73.25(GP19) U73.26(GP20) U73.27(GP21) U73.29(GP22) U73.30(RUN) U73.31(GP26) U73.32(GP27) U73.34(GP28) U73.35(ADC_REF) U73.37(3V3_EN) U73.41(SWCLK) U73.43(SWDIO) U73.BOOTSEL U74.1(GND) U74.2(RF4) U74.3(GND) U74.4(GND) U74.5(GND) U74.6(GND) U74.7(RF2) U74.8(GND) U74.9(GND) U74.10(GND) U74.11(GND) U74.12(GND) U74.13(RFC) U74.14(GND) U74.15(GND) U74.16(GND) U74.17(GND) U74.18(RF1) U74.19(GND) U74.20(GND) U74.21(GND) U74.22(GND) U74.23(RF3) U74.24(GND) U74.25(GND) U74.26(GND) U74.27(VDD) U74.28(GND) U74.29(V1) U74.30(V2) U74.31(GND) U74.32(GND) U74.EP(GND) U75.1(RTN) U75.2(VIN) U75.3(GND) U75.4(VOUT) U76.1(RTN) U76.2(VIN) U76.3(GND) U76.4(VOUT) U77.1(ZR1) U77.2(!MS!/ADR) U77.3(MC/SCL) U77.4(MD/SDA) U77.5(SCK) U77.6(DATA1) U77.7(BCK) U77.8(LRCK) U77.9(VDD) U77.10(DGND) U77.11(DATA2) U77.12(DATA3) U77.13(DATA4) U77.14(MSEL) U77.15(VOUT8) U77.16(VOUT7) U77.17(VCC) U77.18(AGND) U77.19(VOUT6) U77.20(VOUT5) U77.21(VOUT4) U77.22(VOUT3) U77.23(VCC) U77.24(AGND) U77.25(VCOM) U77.26(VOUT2) U77.27(VOUT1) U77.28(ZR2) U77.EP(DGND) U78.1(IN) U78.2(GND) U78.3(OUT) U79.1(OUT) U79.2(IN-) U79.3(IN+) U79.4(-VS) U79.5(IN+) U79.6(IN-) U79.7(OUT) U79.8(+VS) U80.2(IN-) U80.3(IN+) U80.4(-VS) U80.6(OUT) U80.7(+VS) U81.1(GND) U81.2(TRIG) U81.3(OUT) U81.4(RST) U81.5(CV) U81.6(THRS) U81.7(DIS) U81.8(VCC) U82.1(HIN) U82.2(LIN) U82.3(GND) U82.4(LO) U82.5(VCC) U82.6(VSW) U82.7(HO) U82.8(VB) U83.1(BST) U83.2(PWM) U83.3(EN) U83.4(VCC) U83.5(DRVL) U83.6(GND) U83.7(SW) U83.8(DRVH) U84.1(IN) U84.2(EN) U84.4(GND) U84.5(OUT) U84.6(ADJ) U84.EP(GND) U85.1(IN) U85.2(GND) U85.3(EN) U85.4(NC) U85.5(OUT) U86.1(AUX_SCK) U86.2(DNC1) U86.3(DNC2) U86.4(GND1) U86.5(VDDA) U86.6(!RST) U86.7(VDDIO) U86.8(GND2) U86.9(CS) U86.10(MOSI) U86.11(MISO) U86.12(SCK) U86.13(GND3) U86.14(PSEL0) U86.15(PSEL1) U86.16(SYNC_IN) U86.17(RSVD) U86.18(AUX_RX) U86.19(AUX_TX) U86.20(SYNC_PPS) U86.21(RTS) U86.22(CTS) U86.23(RX/SDA) U86.24(TX/SCL) U86.25(GND4) U86.26(AUX_CS) U86.27(AUX_MOSI) U86.28(AUX_MISO) U87.1(MODE) U87.2(SYNCIN) U87.3(VIN) U87.4(PGND) U87.4A(PGND) U87.5(PGND) U87.6(BST) U87.7(SW) U87.7A(SW) U87.8(SW) U87.9(EN) U87.10(PGND) U87.10A(PGND) U87.11(PGND) U87.12(VIN) U87.13(SYNCO) U87.14(PG) U87.15(ICS) U87.16(VCC) U87.17(AGND) U87.18(FB) U87.19(SS) U87.20(FREQ) U88.2(AGND) U88.3(VDD) U88.4(VDRV) U88.5(PGND) U88.9(PGND) U88.10(SW) U88.20(PGND) U88.29(VIN) U88.30(VIN) U88.32(SW) U88.33(BST) U88.34(PWM) U88.35(EN) U88.36(TOUT) U88.38(IOUT) U88.40(PGND) U89.1(CST) U89.1A(CST) U89.2(VCC) U89.3(TPOR) U89.4(OVP) U89.5(SAS) U89.6(PFI) U89.7(DVDT) U89.8(ILIM) U89.9(AGND) U89.10(DET) U89.10A(DET) U89.11(VIN) U89.12(VB) U89.13(EN) U89.14(VBO) U89.15(PGS) U89.16(PGB) U89.16A(PGB) U89.17(INT) U89.18(SDA) U89.19(SCL) U89.20(TEMP) U89.21(ICH) U89.22(FBB) U89.23(FBS) U89.24(RTEST) U89.25(BST) U89.25A(BST) U89.26(STGR) U89.27(SW) U89.28(PGND) U89.29(VB) U89.30(VIN) U90.1(PGND) U90.2(PGND) U90.3(SW) U90.4(OUT) U90.5(OUT) U90.6(OUT) U90.8(EN) U90.9(IN) U90.10(INA) U90.11(AGND) U90.12(FB) U90.13(PGND) U90.14(SW) U91.1(ILIM) U91.2(PGND) U91.3(SW) U91.4(BST) U91.5(PVIN) U91.6(PVIN) U91.7(PVIN) U91.8(PVIN) U91.9(PVIN) U91.10(PVIN) U91.11(PVIN) U91.12(SW) U91.13(SW) U91.14(SW) U91.15(SW) U91.16(PGND) U91.17(PGND) U91.18(PGND) U91.19(PGND) U91.20(SW) U91.21(PVDD) U91.22(PGND) U91.23(EXTVDD) U91.24(EN) U91.25(FREQ) U91.26(SS) U91.27(FB) U91.28(AGND) U91.29(PGND) U91.30(VDD) U91.31(SVIN) U91.32(PG) U91.PGND U91.PGND2(PGND) U91.PVIN U91.SW U92.1(OUT) U92.2(+VS) U92.3(IN+) U92.4(IN-) U92.5(-VS) U93.1(VDD) U93.2(HB) U93.3(HO) U93.4(HS) U93.5(HI) U93.6(LI) U93.7(VSS) U93.8(LO) U94.1(IN) U94.2(GND) U94.3(OUT) U94.T(GND) U95.1(SW) U95.2(GND) U95.3(FB) U95.4(EN) U95.5(VIN) U96.1(HSD) U96.2(EN) U96.3(FB) U96.4(GND) U96.5(VDD) U96.6(LO) U96.7(PGND) U96.8(HO) U96.9(SW) U96.10(BST) U97.1(IN) U97.2(GND) U97.4(OUT) U97.5(VDD) U98.1(IN) U98.2(GND) U98.3(EN) U98.5(OUT) U99.1(STAT) U99.2(VSS) U99.3(VBAT) U99.4(VDD) U99.5(PROG) U100.1(CE) U100.2(VSS) U100.3(VBAT) U100.4(VDD) U100.5(PROG) U101.1(VDD) U101.2(VDD) U101.3(VBAT) U101.4(VBAT) U101.7(STAT) U101.8(GND) U101.9(GND) U101.10(PROG) U101.GF(GND) U102.1(B0) U102.2(B1) U102.3(B2) U102.4(B3) U102.5(B4) U102.6(B5) U102.7(B6) U102.8(B7) U102.9(VDD) U102.10(VSS) U102.12(SCL) U102.13(SDA) U102.15(AD0) U102.16(AD1) U102.17(AD2) U102.18(RST) U102.19(INTB) U102.20(INTA) U102.21(A0) U102.22(A1) U102.23(A2) U102.24(A3) U102.25(A4) U102.26(A5) U102.27(A6) U102.28(A7) U103.1(VIN) U103.2(VOUT) U103.3(GND) U104.1(OUT) U104.2(-VS) U104.3(IN+) U104.4(IN-) U104.5(+VS) U105.1(OUT) U105.2(-) U105.3(+) U105.4(VCC) U105.5(+) U105.6(-) U105.7(OUT) U105.8(OUT) U105.9(-) U105.10(+) U105.11(VSS) U105.12(+) U105.13(-) U105.14(OUT) U106.1(OUT) U106.2(IN-) U106.3(IN+) U106.4(-VS) U106.5(IN+) U106.6(IN-) U106.7(OUT) U106.8(+VS) U107.1(OUT) U107.2(GND) U107.3(VCC) U107.4(SDA) U107.5(SCL) U107.6(ADR) U108.1(GND) U108.2(OUT) U108.3(IN) U109.0(GND) U109.1(GND) U109.2(GND) U109.3(GND) U109.4(VFB) U109.5(MODE) U109.6(VIN) U109.7(EN) U109.8(SW) U109.9(SW) U109.10(GND) U110.1(COMP) U110.2(FB) U110.3(CS) U110.4(EN) U110.5(GND) U110.6(VOUT) U110.7(VCC) U110.8(VREF) U111.1(V+) U111.2(IN) U111.4(GND) U111.5(GND) U111.6(OUT) U111.7(OUT) U111.8(V+) U112.1(OUT) U112.2(-VS) U112.3(IN+) U112.4(IN-) U112.5(+VS) U113.1(Q3) U113.2(Q0) U113.3(R0) U113.4(S0) U113.5(EN) U113.6(S1) U113.7(R1) U113.8(GND) U113.9(Q1) U113.10(Q2) U113.11(R2) U113.12(S2) U113.13(NC) U113.14(S3) U113.15(R3) U113.16(VCC) U114.1(Q3) U114.2(Q0) U114.3(R0) U114.4(S0) U114.5(EN) U114.6(S1) U114.7(R1) U114.8(GND) U114.9(Q1) U114.10(Q2) U114.11(R2) U114.12(S2) U114.13(NC) U114.14(S3) U114.15(R3) U114.16(VCC) U115.1(A0) U115.2(B0) U115.3(O0) U115.4(A1) U115.5(B1) U115.6(O1) U115.7(GND) U115.8(O3) U115.9(B3) U115.10(A3) U115.11(O2) U115.12(B2) U115.13(A2) U116.1(OUT) U116.2(-) U116.3(+) U116.4(VSS) U116.5(+) U116.6(-) U116.7(OUT) U116.8(VCC) U117.1(OUT) U117.2(OUT) U117.3(+VS) U117.4(IN-) U117.5(IN+) U117.6(IN-) U117.7(IN+) U117.8(IN-) U117.9(IN+) U117.10(IN-) U117.11(IN+) U117.12(-VS) U117.13(OUT) U117.14(OUT) U118.1(IN) U118.2(EN) U118.3(GND) U118.4(SET) U118.5(SNS) U118.6(OUT) U118.EP(GND) U119.1(C1+) U119.2(VS+) U119.3(C1-) U119.4(C2+) U119.5(C2-) U119.6(VS-) U119.7(T2OUT) U119.8(R2IN) U119.9(R2OUT) U119.10(T2IN) U119.11(T1IN) U119.12(R1OUT) U119.13(R1IN) U119.14(T1OUT) U119.15(GND) U119.16(VCC) U120.1(LO) U120.2(GND) U120.3(RFIN) U120.4(IFOUT) U120.5(VCC) U120.6(!SHDN) U121.1(LO) U121.2(GND) U121.3(IF) U121.4(RF) U121.5(VCC) U121.6(!SHDN) U122.1(LO) U122.2(GND) U122.3(IFIN) U122.4(RFOUT) U122.5(VCC) U122.6(!SHDN) U123.1(C1+) U123.2(VS+) U123.3(C1-) U123.4(C2+) U123.5(C2-) U123.6(VS-) U123.7(T2OUT) U123.8(R2IN) U123.9(R2OUT) U123.10(T2IN) U123.11(T1IN) U123.12(R1OUT) U123.13(R1IN) U123.14(T1OUT) U123.15(GND) U123.16(VCC) U124.1(GND1) U124.2(TXD) U124.3(RXD) U124.4(PPS) U124.5(EXTINT) U124.6(V_BCKP) U124.7(VCC_IO) U124.8(VCC) U124.9(RESET_IN) U124.10(GND2) U124.11(RF_IN) U124.12(GND3) U124.13(LNA_EN) U124.14(VCC_RF) U124.15(V_ANT) U124.16(SDA) U124.17(SCL) U124.18(SAFEBOOT_N) U125.1 U125.2 U125.3 U125.4 U125.5 U125.6 U125.7 U125.8 U126.1 U126.2 U126.3 U126.4 U127.1(TRIG) U127.2(GND) U127.3(SET) U127.4(DIV) U127.5(V+) U127.6(OUT) U128.1(MOD) U128.2(GND) U128.3(SET) U128.4(DIV) U128.5(V+) U128.6(OUT) U129.1(OE) U129.2(GND) U129.3(SET) U129.4(DIV) U129.5(V+) U129.6(OUT) U130.P1(VIN) U130.P2(UV) U130.P3(OV) U130.P4(GND) U130.P5(!SHDN) U130.P6(!FAULT) U130.P7(VOUT) U130.P8(GATE) U131.1(!SHDN) U131.2(VCC) U131.3(GND) U131.4(SW) U131.5(VOUT) U131.6(CAP) U131.7(VREF) U131.8(FB) U131.GF(GND) U132.1(GND) U132.2(GND) U132.4(VIN) U132.6(VREF) U133.1(OUT) U133.2(OUT) U133.3(OUT) U133.4(SET) U133.7(IN) U133.8(IN) U133.GF(OUT) U134.1(SET) U134.2(OUT) U134.3(IN) U134.T(OUT) U135.2(NC_2) U135.3(OUT_2) U135.4(OUT) U135.5(ADJ) U135.7(NC_3) U135.10(NC_4) U135.11(!SHDN) U135.12(NC_5) U135.13(IN_2) U135.14(IN) U135.15(NC) U135.EPAD U136.1(OUT) U136.2(IN-) U136.3(IN+) U136.4(-VS) U136.5(IN+) U136.6(IN-) U136.7(OUT) U136.8(+VS) U137.3(FB) U137.4(CAP+) U137.5(GND) U137.6(CAP-) U137.11(VOUT) U137.12(VREF) U137.13(OSC) U137.14(VCC) U138.1(VIN) U138.2(CHG) U138.3(PG) U138.4(EN) U138.5(NTC) U138.6(GND) U138.7(NC) U138.8(IBF) U138.9(ISET) U138.10(BAT) U138.GF(GND) U139.1(OUT) U139.2(-VS) U139.3(IN+) U139.4(IN-) U139.5(EN) U139.6(+VS) U140.1(IN+) U140.2(-VS) U140.3(IN-) U140.4(OUT) U140.5(+VS) U141.1(VOUT) U141.2(GND) U141.3(VIN) U142.1(GND) U142.2(EN) U142.3(VIN) U142.4(RT) U142.5(FB) U142.6(PG) U142.7(BOOT) U142.8(SW) U142.TP(GND) U143.1(OUT) U143.2(-VS) U143.3(IN+) U143.4(IN-) U143.5(+VS) U144.1(NC) U144.2(C+) U144.3(GND) U144.4(C-) U144.5(VO) U144.6(LV) U144.7(OSC) U144.8(VIN) U145.1(OUT) U145.2(IN-) U145.3(IN+) U145.4(-VS) U145.5(IN+) U145.6(IN-) U145.7(OUT) U145.8(+VS) U146.1(OUT) U146.2(IN-) U146.3(IN+) U146.4(-VS) U146.5(IN+) U146.6(IN-) U146.7(OUT) U146.8(+VS) U147.2(TRIG) U147.3(OUT) U147.4(RESET) U147.5(CV) U147.6(TRSH) U147.7(DISCH) U148.1(SW) U148.2(SW) U148.3(CBOOT) U148.4(VCC) U148.5(BIAS) U148.6(SYNC) U148.7(RT) U148.8(PGOOD) U148.9(FB) U148.10(AGND) U148.11(SS/TRK) U148.12(EN) U148.13(VIN) U148.14(VIN) U148.15(PGND) U148.16(PGND) U148.P$1(PGND) U149.1(VIN) U149.2(UVLO) U149.3(RT) U149.4(EN) U149.5(RAMP) U149.6(AGND) U149.7(SS) U149.8(FB) U149.9(COMP) U149.10(VOUT) U149.11(DEMB) U149.12(CS) U149.13(CSG) U149.14(PGND) U149.15(LO) U149.16(VCC) U149.17(VCCX) U149.18(HB) U149.19(HO) U149.20(SW) U149.TP(PGND) U150.1(OUT) U150.2(-VS) U150.3(IN+) U150.4(IN-) U150.5(+VS) U151.1(BIAS) U151.2(VCC) U151.3(GATE) U151.4(PGND) U151.5(CS) U151.6(COMP) U151.7(AGND) U151.8(FB) U151.9(SS) U151.10(RT) U151.11(PG) U151.12(UVLO) U151.P$13(AGND) U152.1(VDD) U152.2(PILOT) U152.3(OUT) U152.4(VSS) U152.5(INB) U152.6(IN) U153.1(VDD) U153.2(HB) U153.3(HO) U153.4(HS) U153.5(RT1) U153.6(RT2) U153.7(HI) U153.8(LI) U153.9(VSS) U153.10(LO) U154.1(K) U154.2(REF) U154.3(A) U155.1(USBDM2) U155.2(USBDP2) U155.3(USBDM3) U155.4(USBDP3) U155.5(VDD33A) U155.6(NC) U155.7(NC) U155.8(NC) U155.9(NC) U155.10(VDD33A) U155.11(VBUS_DET) U155.12(NRST) U155.13(TEST1) U155.14(PRTCTL2) U155.15(VDD18CORE) U155.16(PRTCTL3) U155.17(NC) U155.18(NC) U155.19(VDD33IO) U155.20(NFDX_LED) U155.21(NLNKA_LED) U155.22(NSPD_LED) U155.23(EECLK) U155.24(EECS) U155.25(EEDO) U155.26(EEDI) U155.27(VDD33IO) U155.28(NTRST) U155.29(TMS) U155.30(TDI) U155.31(TDO) U155.32(TCK) U155.33(VDD33IO) U155.34(TEST2) U155.35(GPIO3) U155.36(GPIO4) U155.37(GPIO5) U155.38(VDD18CORE) U155.39(VDD33IO) U155.40(TEST3) U155.41(AUTOMDIX_EN) U155.42(GPIO6) U155.43(GPIO7) U155.44(CLK24_EN) U155.45(CLK24_OUT) U155.46(VDD33IO) U155.47(TEST4) U155.48(VDD18ETHPLL) U155.49(VDD33A) U155.50(EXTRES) U155.51(VDD33A) U155.52(RXP) U155.53(RXN) U155.54(VDD33A) U155.55(TXP) U155.56(TXN) U155.57(VDD33A) U155.58(USBDM0) U155.59(USBDP0) U155.60(XO) U155.61(XI) U155.62(VDD18USBPLL) U155.63(USBRBIAS) U155.64(VDD33A) U155.P$1(GND) U156.1(VDD2A) U156.2(LED2) U156.3(LED1) U156.4(XTAL2) U156.5(XTAL1/CLKIN) U156.6(VDDCR) U156.7(RXD1) U156.8(RXD0) U156.9(VDDIO) U156.10(RXER/PHYAD0) U156.11(CRS_DV/MODE2) U156.12(MDIO) U156.13(MDC) U156.14(REFCLKO) U156.15(NRST) U156.16(TXEN) U156.17(TXD0) U156.18(TXD1) U156.19(VDD1A) U156.20(TXN) U156.21(TXP) U156.22(RXN) U156.23(RXP) U156.24(RBIAS) U156.EP(VSS) U157.1(~LIN) U157.2(SD/OD) U157.3(HIN) U157.4(VCC) U157.5(DT) U157.6(SGND) U157.7(PGND) U157.8(LOUT) U157.9(CP-) U157.10(CP+) U157.11(NC) U157.12(VSW) U157.13(HOUT) U157.14(BOOT) U158.1(IN) U158.2(GND) U158.3(OUT) U158.T(GND) U159.1(VOUT) U159.2(GND) U159.3(GND) U159.5(SHDN) U159.6(GND) U159.7(GND) U159.8(VIN) U160.1(IN) U160.3(OUT) U160.T(GND) U161.1(IN) U161.2(GND) U161.3(OUT) U162.1(VCC1) U162.2(SDA1) U162.3(SCL1) U162.4(GND1) U162.5(GND2) U162.6(SCL2) U162.7(SDA2) U162.8(VCC2) U163.1(VCC) U163.2(R) U163.3(D) U163.4(GND) U163.5(Y) U163.6(Z) U163.7(B) U163.8(A) U164.1(VIN) U164.2(VREF) U164.3(GND) U165.1(LIN) U165.2(HIN) U165.3(VCC) U165.4(GND) U165.5(LO) U165.6(VSW) U165.7(HO) U165.8(VB) U166.1(VCC) U166.2(HIN) U166.3(LIN) U166.4(GND) U166.5(LO) U166.6(VSW) U166.7(HO) U166.8(VB) U167.+V(5V) U167.-V(GND) U167.AC/L U167.AC/N U168.2(IN+) U168.3(IN-) U168.4(GND) U168.5(VS) U168.6(REF2) U168.7(REF1) U168.8(OUT) U169.1(REF) U169.2(GND) U169.3(VS) U169.4(IN+) U169.5(IN-) U169.6(OUT) U170.1(OUT) U170.2(-VS) U170.3(IN+) U170.4(IN-) U170.5(+VS) U171.1(OUT) U171.2(GND) U171.3(IN+) U171.4(IN-) U171.5(REF) U171.6(VS) U172.1(OUT) U172.2(GND) U172.3(IN+) U172.4(IN-) U172.5(VS) U173.P2_1(GND) U173.P2_2(VS) U173.P2_3(VDD) U173.P2_4(VEXT) U173.P2_5(GND2) U173.P2_6(SCL) U173.P2_7(SDA) U173.P2_8(GPIO0) U173.P2_9(GPIO5) U173.P2_10(GPIO4) U173.P2_11(RESET) U173.P3_1(GND1) U173.P3_2(VIN) U173.P3_3(MOSI) U173.P3_4(MISO) U173.P3_5(SCK) U173.P3_6(TXD) U173.P3_7(RXD) U173.P3_8(GPIO3) U173.P3_9(GPIO2) U173.P3_10(GPIO1) U173.P3_11(ADC) U174.1(RF2) U174.2(GND) U174.3(RF1) U174.4(B) U174.5(RFC) U174.6(A) U175.15(GND) U175.16(RFOUT) U175.20(VCC) U175.22(VTUNE) U175.EP(GND) U176.J2_1(GND1) U176.J2_2(5V) U176.J2_3(VEXT1) U176.J2_4(VEXT2) U176.J2_5 U176.J2_6 U176.J2_7(CHIP_PU) U176.J2_8(USER_KEY) U176.J2_9 U176.J2_10 U176.J2_11 U176.J2_12 U176.J2_13 U176.J2_14 U176.J2_15 U176.J2_16 U176.J2_17 U176.J2_18 U176.J3_1(GND2) U176.J3_2(3V3_1) U176.J3_3(3V3_2) U176.J3_4 U176.J3_5 U176.J3_6 U176.J3_7 U176.J3_8 U176.J3_9 U176.J3_10 U176.J3_11 U176.J3_12 U176.J3_13 U176.J3_14 U176.J3_15 U176.J3_16 U176.J3_17 U176.J3_18 U177.1(B:2Y0) U177.2(B:2Y2) U177.3(B:2COM) U177.4(B:2Y3) U177.5(B:2Y1) U177.6(A:INH) U177.7(B:GND) U177.8(B:GND) U177.9(A:B) U177.10(A:A) U177.11(A:1Y3) U177.12(A:1Y0) U177.13(A:1COM) U177.14(A:1Y1) U177.15(A:1Y2) U177.16(B:VCC) U178.1(GND1) U178.2(A0+) U178.3(A0-) U178.4(GND2) U178.5(VDD1) U178.6(A1+) U178.7(A1-) U178.8(NC1) U178.9(SEL) U178.10(GND3) U178.11(A2+) U178.12(A2-) U178.13(VDD2) U178.14(GND4) U178.15(A3+) U178.16(A3-) U178.17(GND5) U178.18(NC2) U178.19(GND6) U178.20(VDD3) U178.21(GND7) U178.22(C3-) U178.23(C3+) U178.24(C2-) U178.25(C2+) U178.26(B3-) U178.27(B3+) U178.28(B2+) U178.29(B2-) U178.30(VDD4) U178.31(C1-) U178.32(C1+) U178.33(C0-) U178.34(C0+) U178.35(B1-) U178.36(B1+) U178.37(B0-) U178.38(B0+) U178.39(GND8) U178.40(VDD5) U178.41(GND9) U178.42(NC3) U178.P$1(GND10) U179.1(VCCA) U179.2(B0) U179.3(A0) U179.4(B1) U179.5(A1) U179.6(B2) U179.7(A2) U179.8(GND) U179.9(A3) U179.10(B3) U179.11(A4) U179.12(B4) U179.14(A5) U179.15(B5) U179.16(VCCB) U180.D(RF_OUT) U180.G(RF_IN) U180.S(GND) U181.1(TXD) U181.2(DTR#) U181.3(RTS#) U181.5(RXD) U181.6(RI#) U181.8(NC1) U181.9(DSR#) U181.10(DCD#) U181.11(CTS#) U181.12(CBUS4) U181.13(CBUS2) U181.14(CBUS3) U181.15(USBDP) U181.16(USBDM) U181.19(RESET#) U181.22(CBUS1) U181.23(CBUS0) U181.24(NC2) U181.26(TEST) U181.27(OSCI) U181.28(OSCO) U182.1(OD) U182.2(CS) U182.3(OC) U182.5(VDD) U182.6(VSS) U183.1(VDD) U183.2(GND) U183.3(IN+) U183.4(LDO) U183.5(OUT) U184.1(VDD) U184.2(GND) U184.3(IN) U184.4(XREF) U184.5(OUT) U185.1(FBP) U185.2(IN+) U185.3(REF) U185.4(FBN) U185.5(OUT-) U185.6(VS+) U185.7(VS-) U185.8(OUT+) U186.1(IN) U186.2(T2) U186.3(T4) U186.4(GND) U186.5(T5) U186.6(T3) U186.7(T1) U186.8(VCC) U187.1(GND) U187.2(VQ) U187.3(VDD) U188.1(IPROPI) U188.2(IN2) U188.3(IN1) U188.4(VREF) U188.5(VM) U188.6(OUT1) U188.7(GND) U188.8(OUT2) U188.TP(GND) U189.1(RX_D3) U189.2(TX_CLK) U189.3(TX_EN/TX_CTRL) U189.4(TX_D0) U189.5(TX_D1) U189.6(TX_D2) U189.7(TX_D3) U189.8(!INT/PWDN) U189.9(RD_M) U189.10(RD_P) U189.11(TD_M) U189.12(TD_P) U189.13(NC1) U189.14(AVD) U189.15(NC2) U189.16(RBIAS) U189.17(LED_0) U189.18(!RESET\) U189.19(MDIO) U189.20(MDC) U189.21(VDDIO) U189.22(XO) U189.23(XI) U189.24(LED1/GPIO1) U189.25(RX_CLK) U189.26(RX_DV/RX_CTRL) U189.27(CRS/CRS_DV) U189.28(RX_ER) U189.29(COL/GPIO2) U189.30(RX_D0) U189.31(RX_D1) U189.32(RX_D2) U189.EP(GND) U190.1(DVDD_1.0) U190.2(CEXT) U190.3(VDDA) U190.4(TX+) U190.5(RX+) U190.6(RX-) U190.7(TX-) U190.8(GPIO2) U190.9(XO) U190.10(XI/50M) U190.11(MDIO) U190.12(MDC) U190.13(RX_D3) U190.14(RX_D2) U190.15(RX_D1) U190.16(RX_D0) U190.17(VDDIO) U190.18(RX_DV/CRS_DV) U190.19(RX_CLK/50M_RMII) U190.20(RX_ER) U190.21(PWDN/INT) U190.22(TX_CLK) U190.23(TX_EN) U190.24(TX_D0) U190.25(TX_D1) U190.26(TX_D2) U190.27(TX_D3) U190.28(LED2/TX_ER) U190.29(LED_0) U190.30(CLKOUT/LED_1) U190.31(!RST_N) U190.32(GPIO1) U190.EP(GND) U191.1(OUT) U191.2(GND) U191.3(VCC) U191.4(SCL) U191.5(SDA) U191.6(ADR) U192.1(EN) U192.2(GND) U192.3(OUT) U192.4(VCC) U193.1(NC) U193.2(GND) U193.3(OUT) U193.4(VCC) U194.1(SPDIFIO) U194.2(DW) U194.3(DR) U194.4(SK) U194.5(CS) U194.6(MUTER) U194.7(PWRSEL) U194.8(XI) U194.9(XO) U194.10(MODE) U194.11(GPIO2) U194.12(LED0) U194.13(GPIO3) U194.14(DVSS1) U194.15(GPIO4) U194.16(SDIN) U194.17(ADSCLK) U194.18(MUTEP) U194.19(ADLRCK) U194.20(ADMCLK) U194.21(LEDR) U194.22(ADSEL) U194.23(TEST) U194.24(AVSS1) U194.25(VBIAS) U194.26(VREF) U194.27(MICIN) U194.28(VSEL) U194.29(AVDD1) U194.30(LOL) U194.31(LOBS) U194.32(LOR) U194.33(AVSS2) U194.34(AVDD2) U194.35(DVDD) U194.36(DVSS2) U194.37(REGV) U194.38(MSEL) U194.39(VOLUP) U194.40(PDSW) U194.41(USBDP) U194.42(USBDM) U194.43(GPIO1) U194.44(SDOUT) U194.45(DAMCLK) U194.46(DALRCK) U194.47(DASCLK) U194.48(VOLDN) U195.1(SEL) U195.2(A1) U195.3(B1) U195.4(D1) U195.5(A2) U195.6(B2) U195.7(D2) U195.8(GND) U195.9(D3) U195.10(B3) U195.11(A3) U195.12(D4) U195.13(B4) U195.14(A4) U195.15(DIS) U195.16(VCC) U196.1 U196.2 U196.3 U196.4 U196.5 U196.6 U196.7 U196.8(GND) U196.9 U196.10 U196.11 U196.12(TC) U196.13(CLK_EN) U196.14(CLK) U196.15(MR) U196.16(VCC) U197.1(VDD1) U197.2(XSD) U197.3(A0+) U197.4(A0-) U197.5(GND1) U197.6(VDD2) U197.7(A1+) U197.8(A1-) U197.9(SEL) U197.10(VDD3) U197.11(GND2) U197.12(C1-) U197.13(C1+) U197.14(C0-) U197.15(C0+) U197.16(B1-) U197.17(B1+) U197.18(B0-) U197.19(B0+) U197.20(GND3) U197.P$2(GND4) U198.1(VDD) U198.2(AVDD) U198.3(VC5) U198.4(VC4) U198.5(VC3) U198.6(VC2) U198.7(VC1) U198.8(AVSS) U198.9(SRP) U198.10(SRN) U198.11(DSG) U198.12(CHGU) U198.13(CHG) U198.14(LD) U198.15(TS) U198.16(VTB) U198.17(CCFG) U198.18(CTRC) U198.19(CTRD) U198.20(DVSS) U199.1(ACN) U199.2(ACP) U199.3(!ACDRV) U199.4(CE) U199.5(STAT1) U199.6(TS) U199.7(TTC) U199.8(PG) U199.9(STAT2) U199.10(VREF) U199.11(ISET1) U199.12(VFB) U199.13(SRN) U199.14(SRP) U199.15(ISET2) U199.16(ACSET) U199.17(GND) U199.18(REGN) U199.19(LODRV) U199.20(PH) U199.21(HDRV) U199.22(BST) U199.23(!BATDRV) U199.24(VCC) U199.EP(GND) U200.1(SW1) U200.2(PVCC1) U200.3(PVCC2) U200.4(AVCC) U200.5(ACN) U200.6(ACP) U200.7(CMSRC) U200.8(ACDRV) U200.9(STAT) U200.10(TS) U200.11(TTC) U200.12(VREF) U200.13(ISET) U200.14(FB) U200.15(SRN) U200.16(SRP) U200.17(ACSET) U200.18(OVPSET) U200.19(!BATDRV) U200.20(REGN) U200.21(BTST) U200.22(GND1) U200.23(GND2) U200.24(SW2) U200.PG(GND1) U201.2(GND) U201.3(VDD) U201.4(BOOTN) U201.5(PS1) U201.6(PS0/WAKE) U201.9(CAP) U201.10(CLKSEL0) U201.11(NRST) U201.14(H_INTN) U201.15(S_SCL) U201.16(S_SDA) U201.17(H_SA0/MOSI) U201.18(H_CSN) U201.19(H_SCL/MISO/RX) U201.20(H_SDA/MISO/TX) U201.25(GNDIO) U201.26(CLKSEL/OUT32) U201.27(XIN32) U201.28(VDDIO) U202.1(GND1) U202.2(CSB) U202.3(SDI/SDA) U202.4(SCK/SCL) U202.5(SDO/ADD) U202.6(VDDIO) U202.7(GND2) U202.8(VDD) U203.1(VCC) U203.2(IN) U203.6(SHDN) U203.7(OUT) U203.EP(GND) U204.1(VCC) U204.3(IN) U204.4(OUT) U204.5(EN) U204.6(R) U204.EP(GND) U205.1(VCC) U205.2(BIAS) U205.3(RF-IN) U205.4(RF-OUT) U205.5(EN) U205.6(I-ADJ) U205.PG(GND) U206.1(VS) U206.2(GND) U206.3(RF_OUT) U206.4(GND) U206.5(GND) U206.6(RF_IN) U207.1(VCC) U207.2(GND) U207.3(OUT) U207.4(GND) U207.5(GND) U207.6(IN) U208.1(IN) U208.2(GND) U208.3(VCC) U208.4(OUT) U209.1(PGND) U209.2(VIN) U209.3(AGND) U209.4(FB) U209.5(COMP) U209.6(EN) U209.7(SW1) U209.8(SW2) U209.TP(PGND) U210.1 U210.2(GND) U210.3(GND) U210.4 U210.5(GND) U211.1(GND) U211.2 U211.3(GND) U211.4(GND) U211.5 U211.6(GND) U212.1(VDD_ANA1) U212.2(GND1) U212.3(ANTP) U212.4(ANTN) U212.5(ANTP1) U212.6(GND2) U212.7(VDD_ANA2) U212.8(FILT) U212.9(L2) U212.10(L1) U212.11(DATA) U212.12(DCLK) U212.13(SYSCLK) U212.14(SEL) U212.15(CLK) U212.16(MISO) U212.17(MOSI) U212.18(NC) U212.19(IRQ) U212.20(PWRAMP) U212.21(ANTSEL) U212.22(NC1) U212.23(VDD_IO) U212.24(NC3) U212.25(GPADC1) U212.26(GPADC2) U212.27(CLK16N) U212.28(CLK16P) U212.P$29(GND1) U213.1(PB5) U213.2(PB3) U213.3(PB4) U213.4(GND) U213.5(PB0) U213.6(PB1) U213.7(PB2) U213.8(VCC) U214.1(TXD) U214.2(GND) U214.3(VCC) U214.4(RXD) U214.5(NSIL) U214.6(CANL) U214.7(CANH) U214.8(STBY) U215.1(GND) U215.2(GND) U215.3(RF_IN) U215.4(VS) U215.5(EN) U215.6(RF_OUT) U216.1(EN) U216.2(FB) U216.3(VREG5) U216.4(SS) U216.5(GND) U216.6(SW) U216.7(BST) U216.8(VIN) U216.TP(GND) U217.1(S1) U217.2(VSS) U217.3(VDD) U217.5(VM) U217.6(S2) U217.EP U218.1(GND) U218.2(OUT) U218.3(IN) U218.T(OUT) U219.1(GND) U219.2(OUT) U219.3(IN) U219.T(OUT) U220.1(GND) U220.2(OUT) U220.3(IN) U220.T(OUT) U221.1(LX) U221.2(BS) U221.3(GND) U221.4(FSW) U221.5(COMP) U221.6(FB) U221.7(SS) U221.8(EN) U221.TP(VIN) U222.1(GND) U222.2(OUT) U222.3(IN) U222.T(OUT) U223.1(RING) U223.2(TIP) U223.3(F/R) U223.4(RM) U223.5(SHK) U223.9(VIN) U223.10(VOUT) U223.11(VA) U223.12(GND) U223.13(VPWR) U223.14(PD) U224.1(ADDR) U224.2(ALERT) U224.3(GND) U224.4(AIN0) U224.5(AIN1) U224.6(AIN2) U224.7(AIN3) U224.8(VDD) U224.9(SDA) U224.10(SCL) U225.1(IN) U225.2(GND) U225.3(EN) U225.4(ADJ) U225.5(OUT) U226.1(IN1) U226.2(D1) U226.3(S1) U226.5(GND) U226.6(S4) U226.7(D4) U226.8(IN4) U226.9(IN3) U226.10(D3) U226.11(S3) U226.13(VDD) U226.14(S2) U226.15(D2) U226.16(IN2) U227.1(CLK) U227.2(DATA) U227.3(LE) U227.4(CE) U227.5(SW) U227.6(VP) U227.7(CP_OUT) U227.8(CPGND) U227.9(AGND) U227.10(AVDD) U227.11(AGND_VCO) U227.12(RF_OUT_A+) U227.13(RF_OUT_A-) U227.14(RF_OUT_B+) U227.15(RF_OUT_B-) U227.16(VVCO) U227.17(VVCO) U227.18(AGND_VCO) U227.19(TEMP) U227.20(VTUNE) U227.21(AGND_VCO) U227.22(RSET) U227.23(VCOM) U227.24(VREF) U227.25(LD) U227.26(PDB_RF) U227.27(DGND) U227.28(DVDD) U227.29(REF_IN) U227.30(MUX_OUT) U227.31(SDGND) U227.32(SVDD) U227.EP(THERM_GND) U228.1(FLO) U228.2(CP) U228.3(CPGND) U228.4(AGND) U228.5(RF_IN-) U228.6(RF_IN+) U228.7(AVDD) U228.8(REF_IN) U228.9(DGND) U228.10(EN) U228.11(CLK) U228.12(DATA) U228.13(LE) U228.14(MUXOUT) U228.15(DVDD) U228.16(VP) U229.1(COM2) U229.2(VPS1) U229.3(PADL) U229.4(INHI) U229.5(INLO) U229.6(PADL) U229.7(COM1) U229.8(ENBL) U229.9(LMDR) U229.10(FLTR) U229.11(PADL) U229.12(LMLO) U229.13(LMHI) U229.14(PADL) U229.15(VPS2) U229.16(VLOG) U230.1(VCC) U230.2(GND) U230.3(VOUT) U230.5(IP+) U230.6(IP-) U231.1(IP1+) U231.2(IP2+) U231.3(IP1-) U231.4(IP2-) U231.5(GND) U231.6(!FAULT) U231.7(VIOUT) U231.8(VCC) U232.1(IP1+) U232.2(IP2+) U232.3(IP1-) U232.4(IP2-) U232.5(GND) U232.6(!FAULT) U232.7(VIOUT) U232.8(VCC) U233.1(VDD1) U233.2(VIN+) U233.3(VIN-) U233.4(GND1) U233.5(GND2) U233.6(VOUT-) U233.7(VOUT+) U233.8(VDD2) U234.1 U234.2 U235.1(Q12) U235.2(Q6) U235.3(Q5) U235.4(Q7) U235.5(Q4) U235.6(Q3) U235.7(Q2) U235.8(GND) U235.9(Q1) U235.10(CLK) U235.11(CLR) U235.12(Q9) U235.13(Q8) U235.14(Q10) U235.15(Q11) U235.16(VCC) U236.1(VCCA) U236.2(1A) U236.3(2A) U236.4(GND) U236.5(DIR) U236.6(2B) U236.7(1B) U236.8(VCCB) U237.1(VCCA) U237.2(DIR) U237.3(A0) U237.4(A1) U237.5(A2) U237.6(A3) U237.7(A4) U237.8(A5) U237.9(A6) U237.10(A7) U237.11(GND) U237.12(GND) U237.13(GND) U237.14(B7) U237.15(B6) U237.16(B5) U237.17(B4) U237.18(B3) U237.19(B2) U237.20(B1) U237.21(B0) U237.22(!OE) U237.23(VCCB) U237.24(VCCB) U238.1(Y4) U238.2(Y6) U238.3(COM) U238.4(Y7) U238.5(Y5) U238.6(INH) U238.7(GND) U238.8(GND) U238.9(C) U238.10(B) U238.11(A) U238.12(Y3) U238.13(Y0) U238.14(Y1) U238.15(Y2) U238.16(VCC) U239.1(IN) U239.2(OUT) U239.3(IN) U239.4(OUT) U239.5(IN) U239.6(OUT) U239.7(-) U239.8(OUT) U239.9(IN) U239.10(OUT) U239.11(IN) U239.12(OUT) U239.13(IN) U239.14(+) U240.1(Y4) U240.2(Y6) U240.3(COM) U240.4(Y7) U240.5(Y5) U240.6(INH) U240.7(GND) U240.8(GND) U240.9(C) U240.10(B) U240.11(A) U240.12(Y3) U240.13(Y0) U240.14(Y1) U240.15(Y2) U240.16(VCC) U$1.P+1(PRI_A) U$1.P+2(PRI_A) U$1.P+3(PRI_A) U$1.P+4(PRI_A) U$1.P+5(PRI_A) U$1.P+6(PRI_A) U$1.P+7(PRI_A) U$1.P+8(PRI_A) U$1.P-1(PRI_B) U$1.P-2(PRI_B) U$1.P-3(PRI_B) U$1.P-4(PRI_B) U$1.P-5(PRI_B) U$1.P-6(PRI_B) U$1.P-7(PRI_B) U$1.P-8(PRI_B) U$1.S+1(SEC_A) U$1.S+2(SEC_A) U$1.S+3(SEC_A) U$1.S+4(SEC_A) U$1.S+5(SEC_A) U$1.S+6(SEC_A) U$1.S-1(SEC_B) U$1.S-2(SEC_B) U$1.S-3(SEC_B) U$1.S-4(SEC_B) U$1.S-5(SEC_B) U$1.S-6(SEC_B) U$1.SC1(SEC_CENTER) U$1.SC2(SEC_CENTER) U$1.SC3(SEC_CENTER) U$1.SC4(SEC_CENTER) U$1.SC5(SEC_CENTER) U$1.SC6(SEC_CENTER) U$2.+(P) U$2.-(N) U$3.P$1 U$3.P$2 U$4.+1 U$4.+2 U$4.-1 U$4.-2 U$5.1(IN) U$5.3(OUT) U$5.T(GND) U$6.1(VCC) U$6.2(IN) U$6.3(GND) U$6.4(GND) U$6.5(EN) U$6.6(GND) U$6.7(OUT) U$6.8(GND) U$6.EP(GND) U$7.1(G) U$7.2(S) U$7.3(D) U$8.A1 U$8.A2 U$9.A1 U$9.A2 U$10.1(VOS) U$10.2(AGND) U$10.3(VDD) U$10.4(VDRV) U$10.5(PGND) U$10.9(PGND) U$10.10(SW) U$10.20(PGND) U$10.29(VIN) U$10.30(VIN) U$10.32(SW) U$10.33(BST) U$10.34(PWM) U$10.35(EN) U$10.36(TOUT) U$10.37(OCSET) U$10.38(IOUT) U$10.39(REFIN) U$10.40(PGND) U$11.1(G) U$11.2(D) U$11.3(S) U$12.1(+VIN) U$12.2(-VIN) U$12.4(-VOUT) U$12.5(NC) U$12.6(+VOUT) U$14.1(IN) U$14.2(GND) U$14.3(EN) U$14.4(OUT) U$14.GF(GND) U$16.1 U$16.2 U$16.3 U$16.4 U$16.5 U$16.6 U$16.7 U$16.8 U$16.9 U$16.10 U$16.11 U$16.12 U$16.13 U$16.14 U$16.15 U$16.16 U$16.17 U$16.18 U$16.19 U$16.20 U$17.1(S1) U$17.3(S2) U$17.7(P2) U$17.8(P1) U$19.1(ANALOG_INPUT) U$19.2(ANALOG_FB) U$19.3(SYLLABIC_FILT_IN) U$19.4(GAIN_CONTROL) U$19.5(REF_IN) U$19.6(FILTER_IN) U$19.7(ANALOG_OUT) U$19.8(VEE) U$19.9(DATA_OUT) U$19.10(VCC/2) U$19.11(!COINCIDENCE) U$19.12(DIG_THRESHOLD) U$19.13(DATA_IN) U$19.14(CLK_IN) U$19.15(ENCODE/!DECODE) U$19.16(VCC) U$20.1(RAMP) U$20.2(UVLO) U$20.3(COMP) U$20.4(FB) U$20.5(RT2) U$20.6(AGND) U$20.7(RT1) U$20.8(CS) U$20.9(RES) U$20.10(SS) U$20.11(PGND) U$20.12(OUTB) U$20.13(OUTA) U$20.14(VCC) U$20.15(REF) U$20.16(VIN) U$21.P$1(VDD) U$21.P$2(PILOT) U$21.P$3(OUT) U$21.P$4(VSS) U$21.P$5(INB) U$21.P$6(IN) U$21.P$7(VSS) U$22.1(IN) U$22.2(GND) U$22.3(OUT) U$22.4(GND) U$22.5(GND) U$22.6(GND) U$23.P$1(G) U$23.P$2(G) U$23.P$3(S) U$23.P$4(S) U$23.P$5(D) U$23.P$6(D) U$23.P$7(D) U$23.P$8(D) U$23.P$9(D) U$23.P$10(S) U$23.P$11(S) U$23.P$12(S) U$23.P$13(S) U$23.P$14(S) U$23.P$15(D) U$23.P$16(D) U$23.P$17(D) U$23.P$18(D) U$23.P$19(D) U$23.P$20(S) U$23.P$21(S) U$23.P$22(S) U$23.P$23(S) U$23.P$24(S) U$24.1 U$24.2(GND) U$24.3 U$24.4(GND) U$25.1 U$25.2 U$25.3 U$25.4 U$25.5 U$25.6 U$25.7 U$25.8 U$26.1(TUNE) U$26.4(BITE) U$26.5(RS232_TX) U$26.6(RS232_RX) U$26.7(VCC) U$26.8(GND) U$26.9(1PPS_IN) U$26.10(1PPS_OUT) U$26.12(RF_OUT) U$27.A1-1 U$27.A1-2 U$27.A2-1 U$27.A2-2 U$27.B1 U$27.B2 U$28.1 U$28.2 U$28.P$1 U$28.P$2 U$28.P$3 U$28.P$4 U$28.P$5 U$28.P$6 U$29.A U$29.C U$30.D(OUT) U$30.G(IN) U$30.S(GND) U$31.1(G) U$31.2(B) U$31.3(C) U$31.4(R) U$32.1(OUT) U$32.2(IN-) U$32.3(IN+) U$32.4(-VS) U$32.5(IN+) U$32.6(IN-) U$32.7(OUT) U$32.8(+VS) U$33.1(INHI) U$33.2(COMM) U$33.3(CLPF) U$33.4(VSET) U$33.5(VOUT) U$33.6(TADJ) U$33.7(VPOS) U$33.8(INLO) U$33.EP(COMM) U$34.P$1 U$34.P$2 U$35.1H U$35.1L U$35.2H U$35.2L U$35.3H U$35.3L U$35.4H U$35.4L U$36.A1 U$36.A2 U$36.B1 U$36.B2 U$37.A1 U$37.A2 U$37.B1 U$37.B2 U$38.P$1 U$39.P+2(P1) U$39.P+3(P1) U$39.P+4(P1) U$39.P+5(P1) U$39.P-1(P2) U$39.P-2(P2) U$39.P-4(P2) U$39.P-5(P2) U$39.S+1(S1) U$39.S+2(S1) U$39.S-1(S2) U$39.S-2(S2) U$40.P$1 U$40.P$2 V1.BL V1.BOT(BOTTOM) V1.BR V1.DOT V1.FIL_M V1.FIL_P V1.GRID_P V1.MID(MIDDLE) V1.NC V1.TL V1.TOP V1.TR VR1.1 VR1.2 VR1.3 VR2.1 VR2.2 VR2.3 VR3.1 VR3.2 VR3.3 VR4.1 VR4.2 VR4.3 VR5.1 VR5.2 VR5.3 X1.A(GND) X1.B X1.C(GND) X1.D(GND) X1.E X1.F(GND) X2.1(GND) X2.2 X2.3(GND) X2.4(GND) X2.5(GND) X2.6(GND) X2.7 X2.8(GND) X2.9(GND) X2.10(GND) X3.1(GND) X3.3(OE) X3.4(VDD) X3.5(OUT) X4.1(GND) X4.3(OE) X4.4(VDD) X4.5(OUT) X5.1(GND) X5.2(GND) X5.3(OUT) X5.4(VCC) X6.1(GND) X6.2(GND) X6.3(OUT) X6.4(VCC) X7.1 X7.2(GND) X7.3 X7.4(GND) X8.P$1 X8.P$2 X9.1 X9.2(GND) X9.3(GND) X9.4 X9.5(GND) X10.1(EN) X10.3(GND) X10.4(OUT) X10.5(!OUT) X10.6(VDD) X11.1 X11.2(GND) X11.3 X11.4(GND) X12.P$1 X12.P$2 X13.P$1 X13.P$2 X14.P$1 X14.P$2 X15.P$1 X15.P$2 Z1.1(GND) Z1.2(IF) Z1.3(RF) Z1.4(GND) Z1.5(GND) Z1.6(LO)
